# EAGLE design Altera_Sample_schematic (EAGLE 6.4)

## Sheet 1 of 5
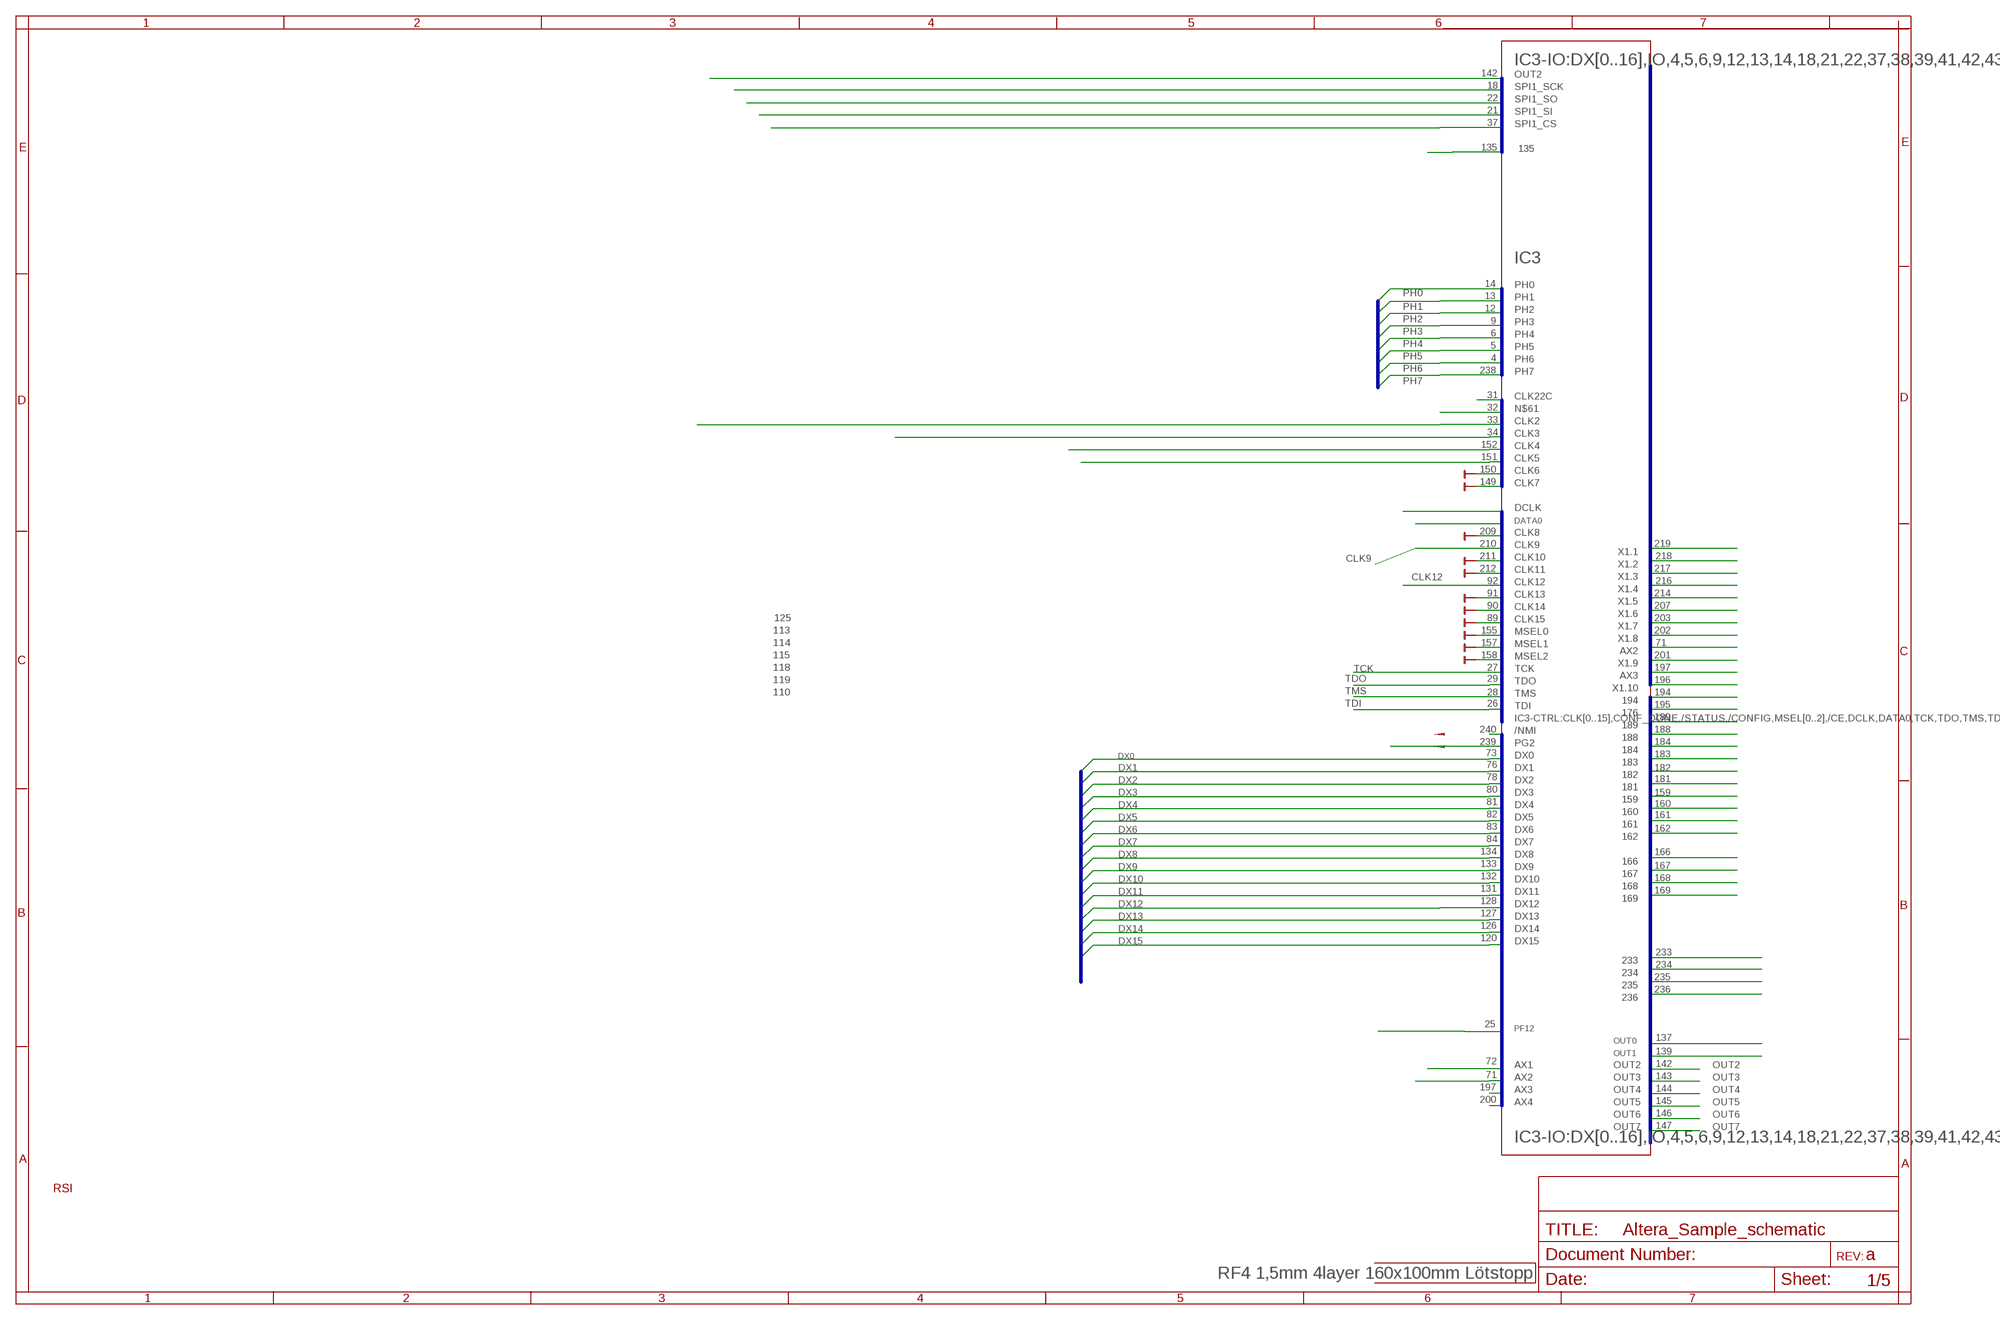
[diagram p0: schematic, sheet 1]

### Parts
PCB  RF4 1,5mm 4layer 160x100mm Lötstopp  PCB  [PCB]

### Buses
DATA:D[0..15]
SPI1:CS,SCK,SI,SO,PH[0..7]
IC3-IO:DX[0..16],IO,4,5,6,9,12,13,14,18,21,22,37,38,39,41,42,43,44,45,46,49,50,51,52,55,56,57,63,64,65,68,69,70,71,72,73,76,78,80,81,82,83,84,87,88,93,94,95,98,99,100,103,106,107,108,109,110,111,112,113,114,117,118,119,120,126,127,128,131,132,133,134,135,137,139,142,148,159,160,161,162,164,166,167,168,169,171,173,176,177,181,182,183,184,185,186,187,188,189,194,195,196,197,200,201,202,203,207,214,216,217,218,219,221,223,224,226,230,231,232,233,234,235,236,237,238,239,240
IC3-CTRL:CLK[0..15],CONF_DONE,/STATUS,/CONFIG,MSEL[0..2],/CE,DCLK,DATA0,TCK,TDO,TMS,TDI
IC3-PH:PH[0..7]

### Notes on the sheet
- 142
- 18
- 22
- 21
- 37
- 135
- IC3
- 14
- 13
- 12
- 9
- 6
- 5
- 4
- 238
- 31
- 32
- 33
- 34
- 152
- 151
- 150
- 149
- 209
- 210 | 219
- 211 | 218
- 212 | 217
- 92 | 216
- 91 | 214
- 90 | 207
- 125 | 89 | 203
- 113 | 155 | 202
- 114 | 157 | 71
- 115 | 158 | 201
- 118 | 27 | 197
- 119 | 29 | 196
- 110 | 28 | 194
- 26 | 195
- 189
- 240 | 188
- 239 | 184
- 73 | 183
- 76
- 182
- 78 | 181
- 80
- 159
- 81 | 160
- 82 | 161
- 83 | 162
- 84
- 134 | 166
- 133 | 167
- 132 | 168
- 131 | 169
- 128
- 127
- 126
- 120
- 233
- 234
- 235
- 236
- 25
- 137
- 139
- 72 | 142
- 71 | 143
- 197 | 144
- 200 | 145
- 146
- 147
- RSI

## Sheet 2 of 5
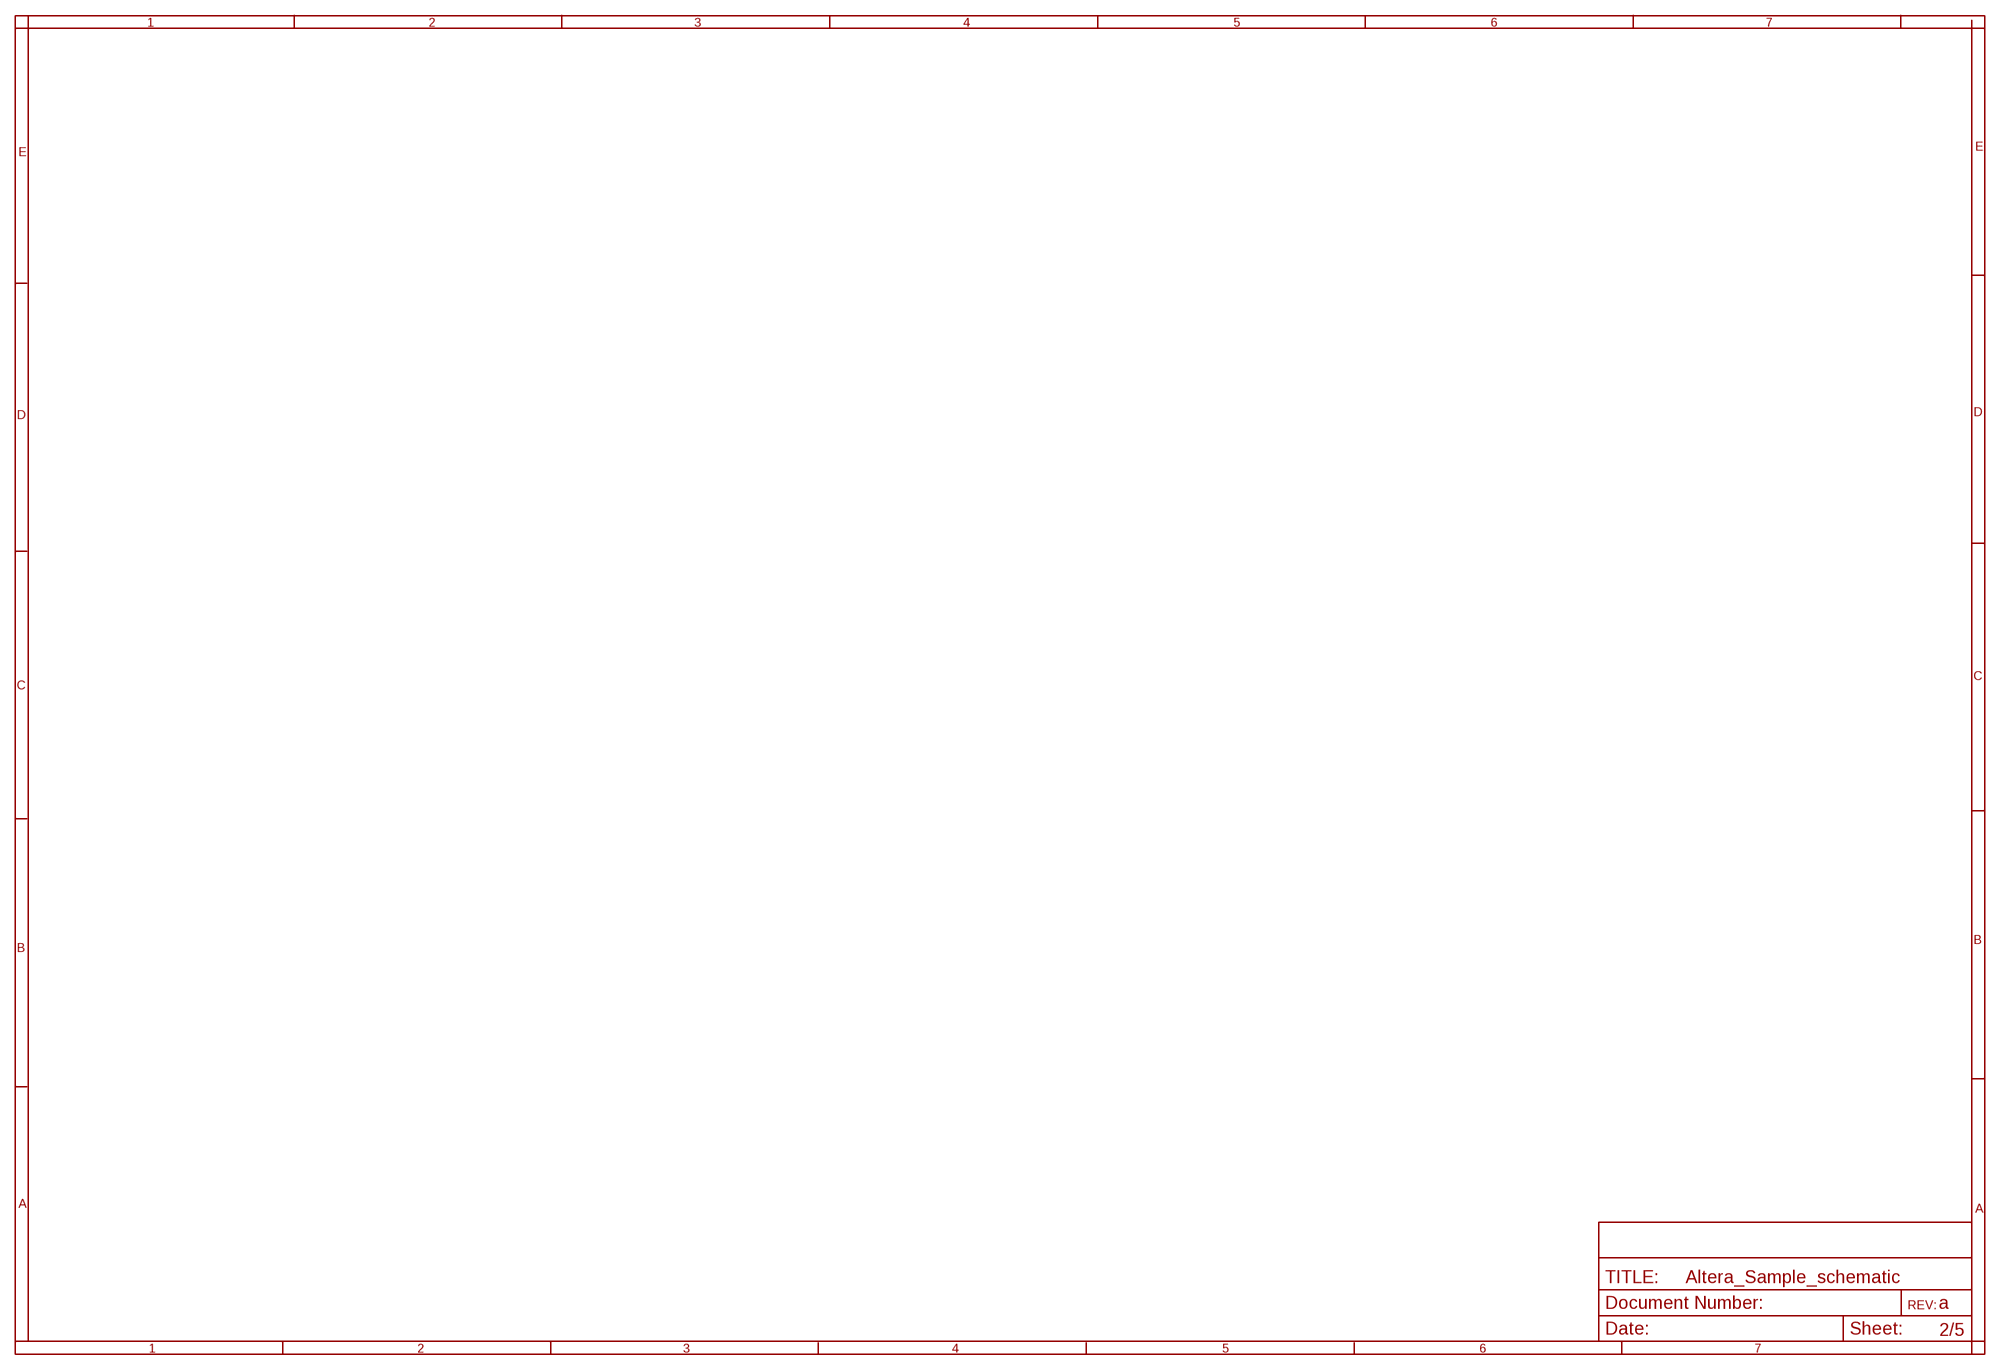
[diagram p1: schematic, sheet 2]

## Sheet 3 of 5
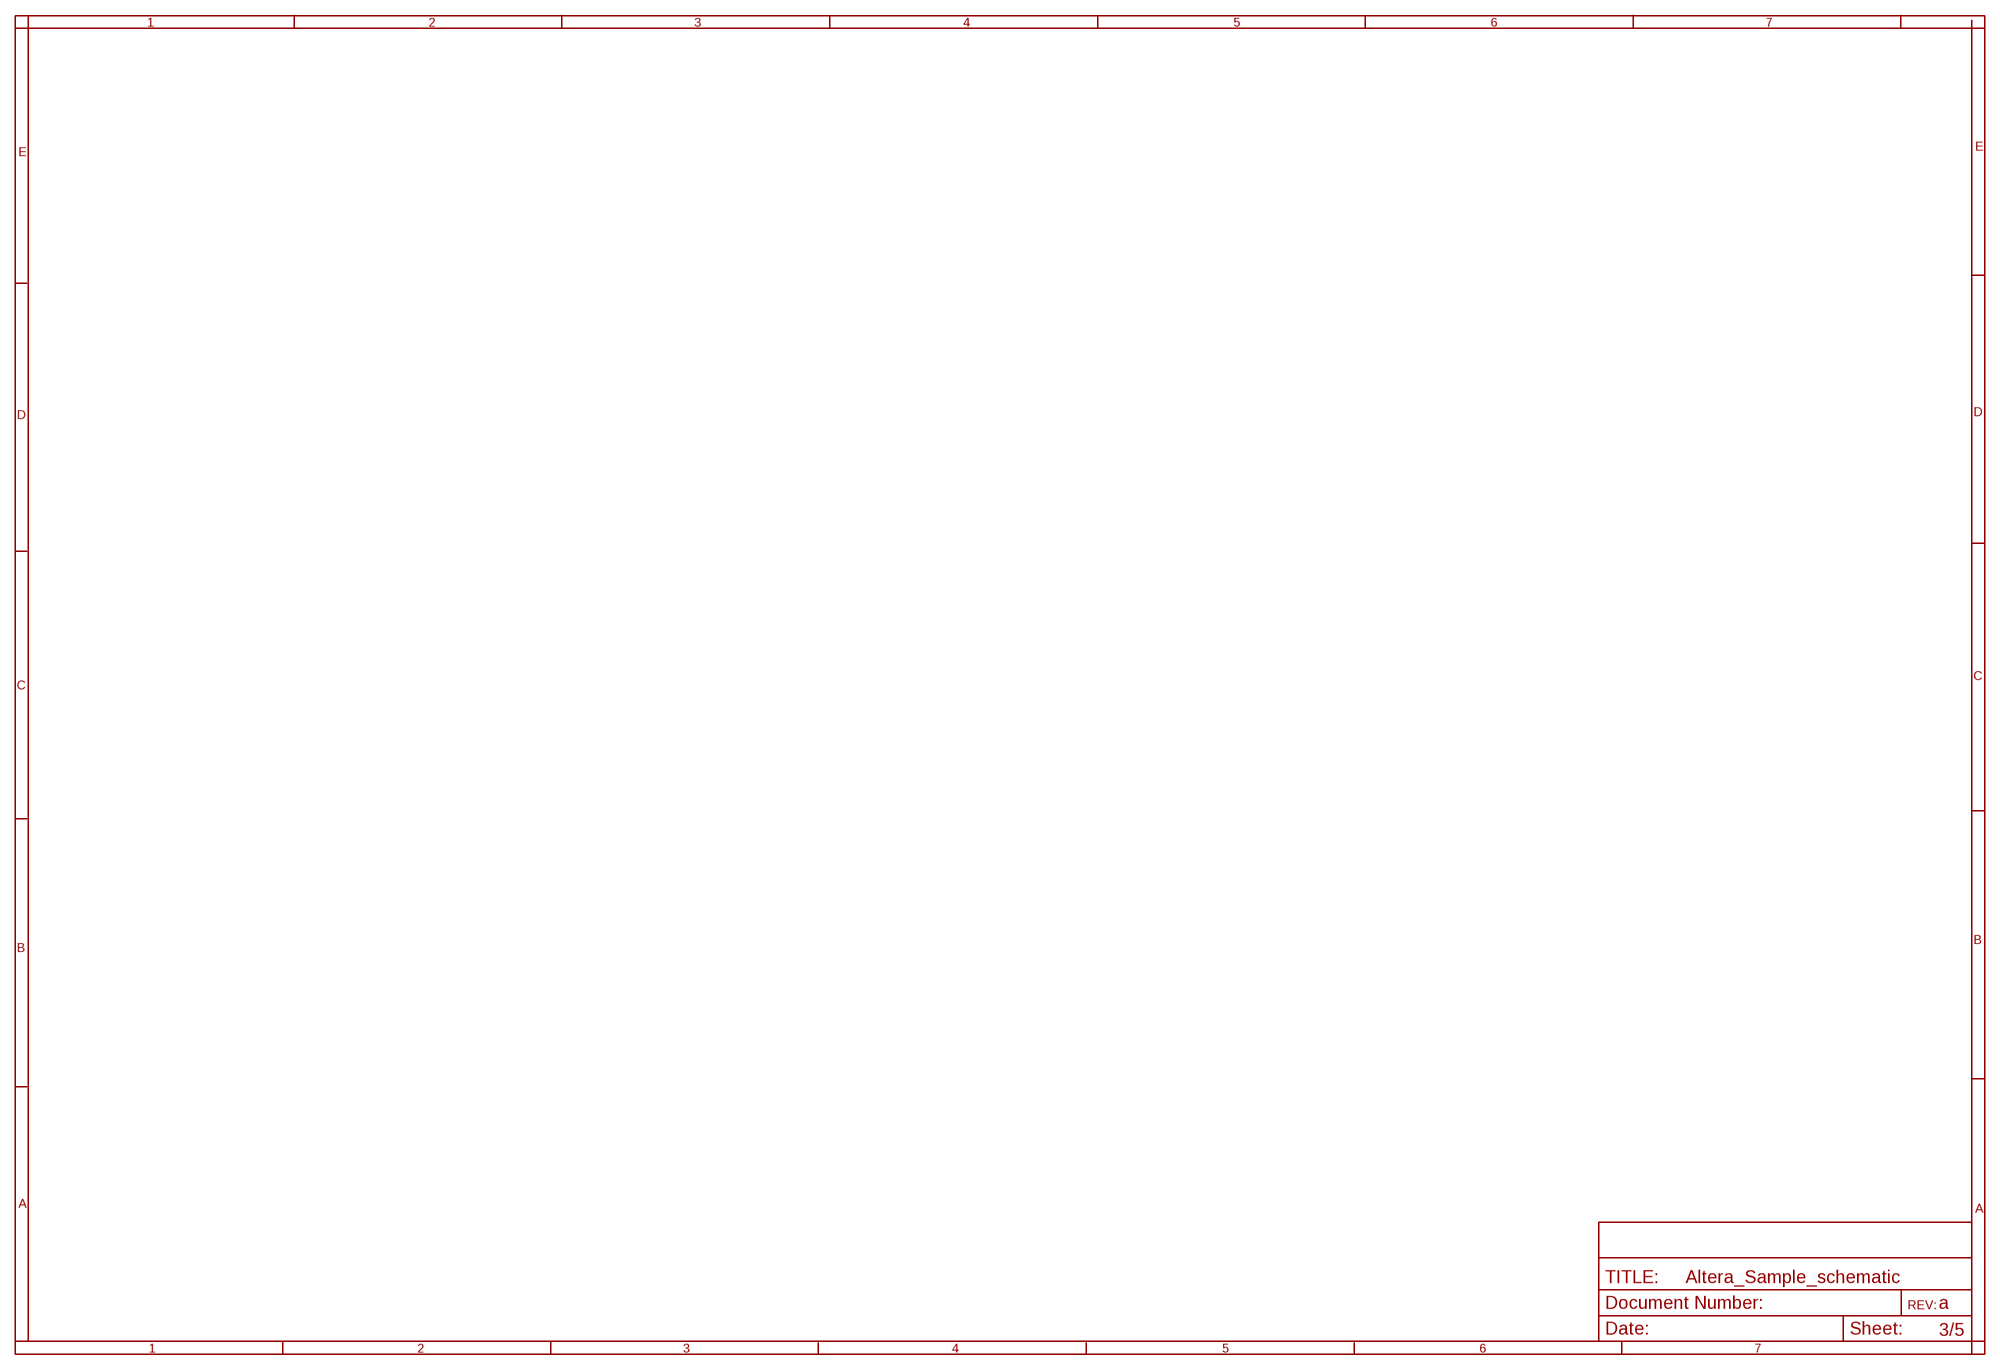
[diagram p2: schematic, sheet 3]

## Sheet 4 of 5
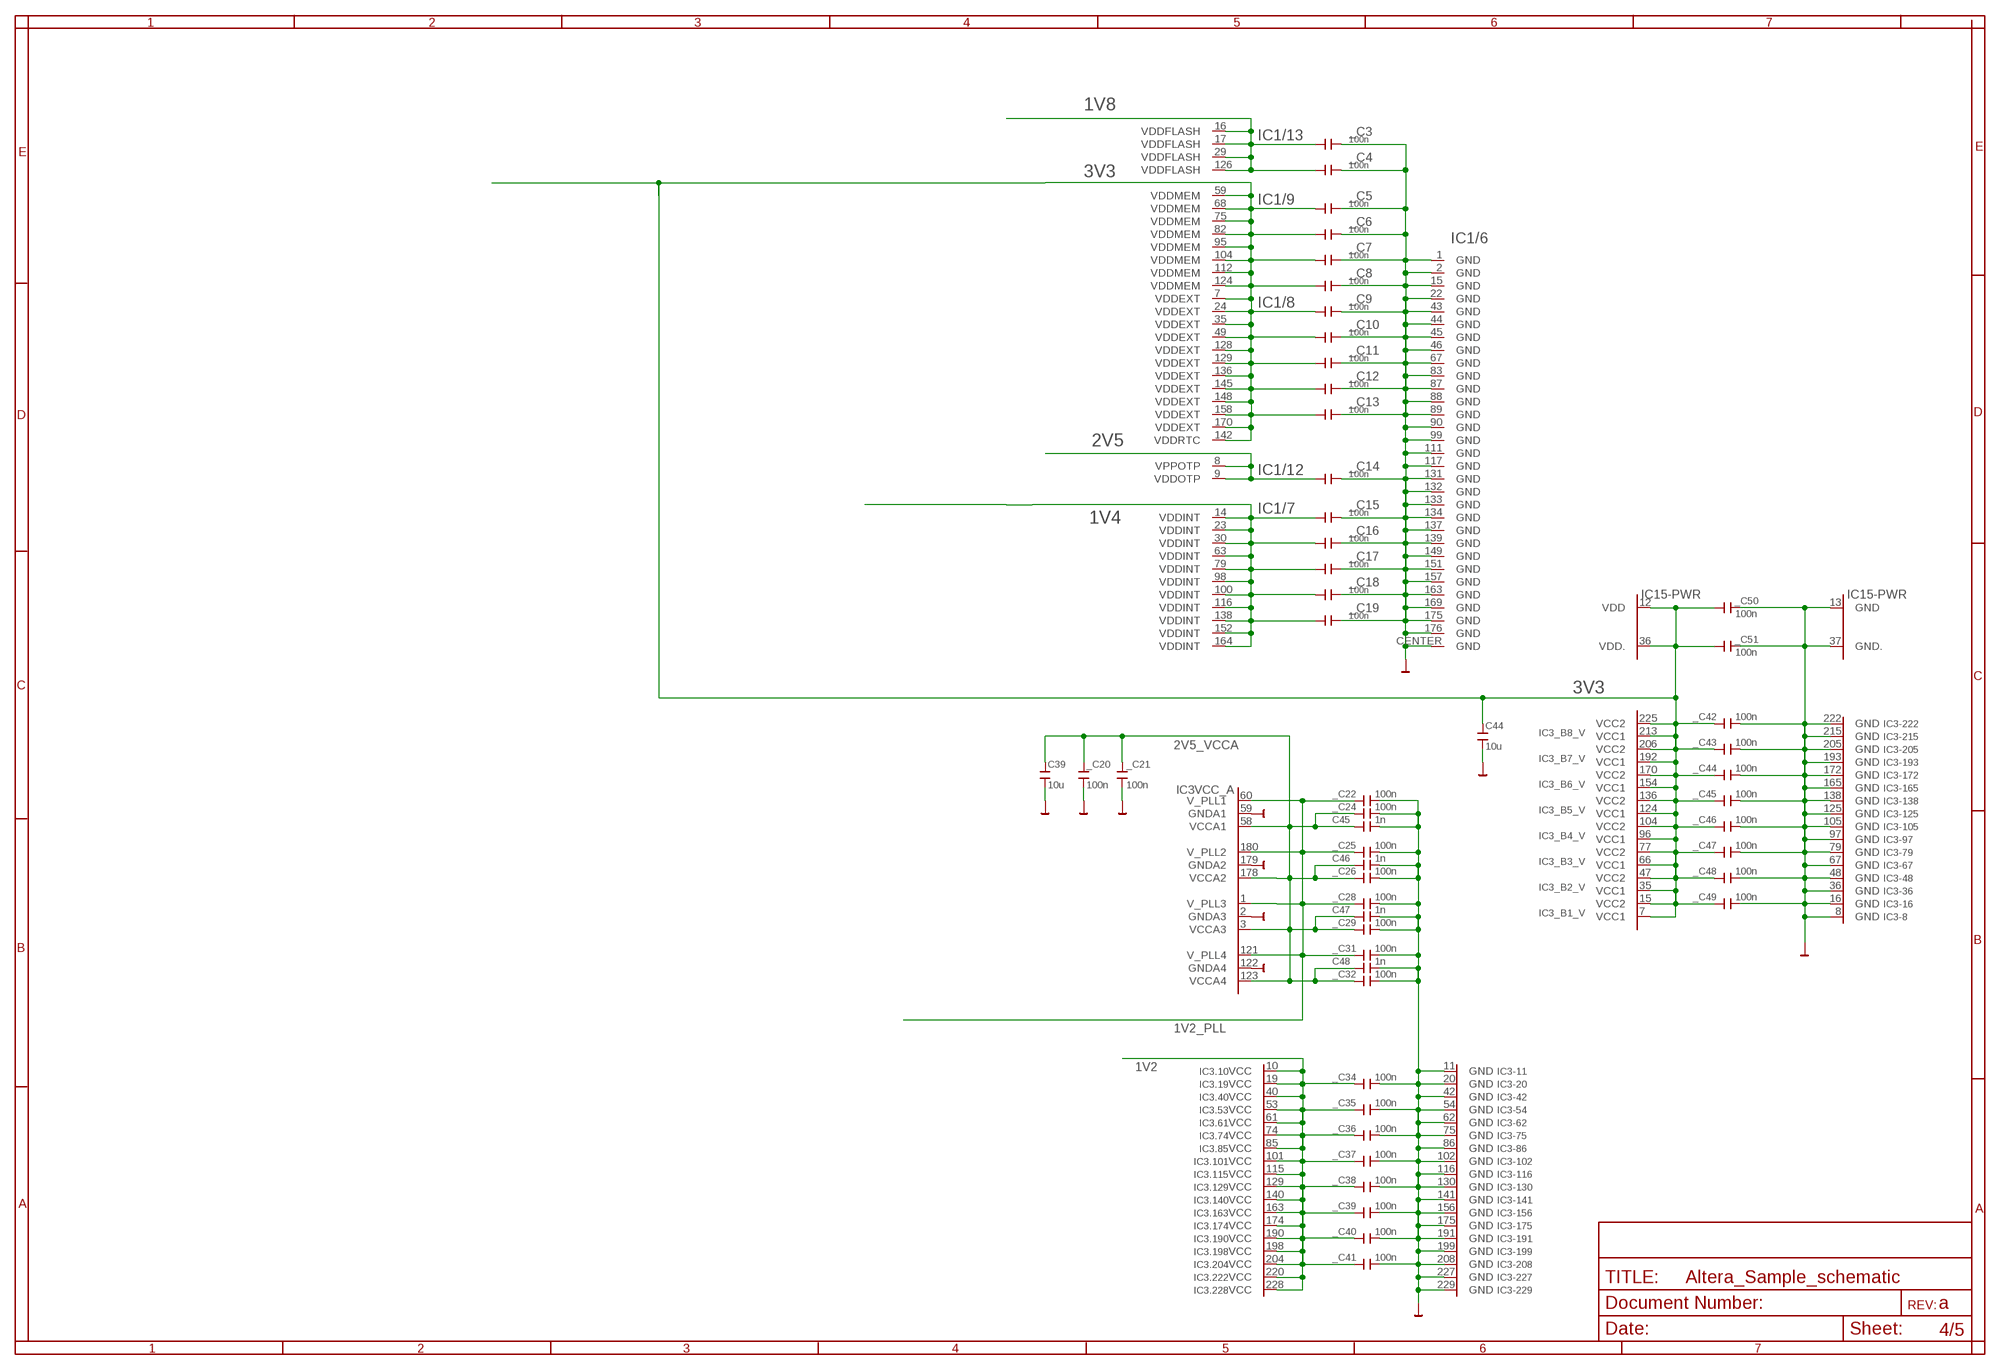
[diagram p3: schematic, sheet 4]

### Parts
_C3  100n  C-EUC0805  [C0805]
_C4  100n  C-EUC0805  [C0805]
_C5  100n  C-EUC0805  [C0805]
_C6  100n  C-EUC0805  [C0805]
_C7  100n  C-EUC0805  [C0805]
_C8  100n  C-EUC0805  [C0805]
_C9  100n  C-EUC0805  [C0805]
_C10  100n  C-EUC0805  [C0805]
_C11  100n  C-EUC0805  [C0805]
_C12  100n  C-EUC0805  [C0805]
_C13  100n  C-EUC0805  [C0805]
_C14  100n  C-EUC0805  [C0805]
_C15  100n  C-EUC0805  [C0805]
_C16  100n  C-EUC0805  [C0805]
_C17  100n  C-EUC0805  [C0805]
_C18  100n  C-EUC0805  [C0805]
_C19  100n  C-EUC0805  [C0805]
_C20  100n  C-EUC0805  [C0805]
_C21  100n  C-EUC0805  [C0805]
_C22  100n  C-EUC0805  [C0805]
_C24  100n  C-EUC0805  [C0805]
_C25  100n  C-EUC0805  [C0805]
_C26  100n  C-EUC0805  [C0805]
_C28  100n  C-EUC0805  [C0805]
_C29  100n  C-EUC0805  [C0805]
_C31  100n  C-EUC0805  [C0805]
_C32  100n  C-EUC0805  [C0805]
_C34  100n  C-EUC0805  [C0805]
_C35  100n  C-EUC0805  [C0805]
_C36  100n  C-EUC0805  [C0805]
_C37  100n  C-EUC0805  [C0805]
_C38  100n  C-EUC0805  [C0805]
_C39  100n  C-EUC0805  [C0805]
_C40  100n  C-EUC0805  [C0805]
_C41  100n  C-EUC0805  [C0805]
_C42  100n  C-EUC0805  [C0805]
_C43  100n  C-EUC0805  [C0805]
_C44  100n  C-EUC0805  [C0805]
_C45  100n  C-EUC0805  [C0805]
_C46  100n  C-EUC0805  [C0805]
_C47  100n  C-EUC0805  [C0805]
_C48  100n  C-EUC0805  [C0805]
_C49  100n  C-EUC0805  [C0805]
_C50  100n  C-EUC0805  [C0805]
_C51  100n  C-EUC0805  [C0805]
C39  10u  C-EUC1210K  [C1210K]
C44  10u  C-EUC1210K  [C1210K]
C45  1n  C-EUC0805  [C0805]
C46  1n  C-EUC0805  [C0805]
C47  1n  C-EUC0805  [C0805]
C48  1n  C-EUC0805  [C0805]
IC1  ADSP-BF514_PART  [LQFP-176+GND]
IC3  EP3C25-Q240-IO131  [PQFP240]
IC15  IS62WV102416ALL  [TSOP1-12X20]

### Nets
1V2: _C34.2 _C35.2 _C36.2 _C37.2 _C38.2 _C39.2 _C40.2 _C41.2 IC3.10(.10:VCC) IC3.19(.19:VCC) IC3.40(.40:VCC) IC3.53(.53:VCC) IC3.61(.61:VCC) IC3.74(.74:VCC) IC3.85(.85:VCC) IC3.101(.101:VCC) IC3.115(.115:VCC) IC3.129(.129:VCC) IC3.140(.140:VCC) IC3.163(.163:VCC) IC3.174(.174:VCC) IC3.190(.190:VCC) IC3.198(.198:VCC) IC3.204(.204:VCC) IC3.220(.222:VCC) IC3.228(.228:VCC)
1V2_PLL: _C22.2 _C25.2 _C28.2 _C31.2 IC3.1(VCC_A:V_PLL3) IC3.60(VCC_A:V_PLL1) IC3.121(VCC_A:V_PLL4) IC3.180(VCC_A:V_PLL2)
1V4: _C15.1 _C16.1 _C17.1 _C18.1 _C19.1 IC1.14(/7:VDDINT) IC1.23(/7:VDDINT) IC1.30(/7:VDDINT) IC1.63(/7:VDDINT) IC1.79(/7:VDDINT) IC1.98(/7:VDDINT) IC1.100(/7:VDDINT) IC1.116(/7:VDDINT) IC1.138(/7:VDDINT) IC1.152(/7:VDDINT) IC1.164(/7:VDDINT)
1V8: _C3.1 _C4.1 IC1.16(/13:VDDFLASH) IC1.17(/13:VDDFLASH) IC1.29(/13:VDDFLASH) IC1.126(/13:VDDFLASH)
2V5: _C14.1 IC1.8(/12:VPPOTP) IC1.9(/12:VDDOTP)
2V5_VCCA: _C20.2 _C21.2 _C24.2 _C26.2 _C29.2 _C32.2 C39.2 C45.2 C46.2 C47.2 C48.2 IC3.3(VCC_A:VCCA3) IC3.58(VCC_A:VCCA1) IC3.123(VCC_A:VCCA4) IC3.178(VCC_A:VCCA2)
3V3: _C5.1 _C6.1 _C7.1 _C8.1 _C9.1 _C10.1 _C11.1 _C12.1 _C13.1 _C42.2 _C43.2 _C44.2 _C45.2 _C46.2 _C47.2 _C48.2 _C49.2 _C50.1 _C51.1 C44.2 IC1.7(/8:VDDEXT) IC1.24(/8:VDDEXT) IC1.35(/8:VDDEXT) IC1.49(/8:VDDEXT) IC1.59(/9:VDDMEM) IC1.68(/9:VDDMEM) IC1.75(/9:VDDMEM) IC1.82(/9:VDDMEM) IC1.95(/9:VDDMEM) IC1.104(/9:VDDMEM) IC1.112(/9:VDDMEM) IC1.124(/9:VDDMEM) IC1.128(/8:VDDEXT) IC1.129(/8:VDDEXT) IC1.136(/8:VDDEXT) IC1.142(/12:VDDRTC) IC1.145(/8:VDDEXT) IC1.148(/8:VDDEXT) IC1.158(/8:VDDEXT) IC1.170(/8:VDDEXT) IC3.7(_B1_V:VCC1) IC3.15(_B1_V:VCC2) IC3.35(_B2_V:VCC1) IC3.47(_B2_V:VCC2) IC3.66(_B3_V:VCC1) IC3.77(_B3_V:VCC2) IC3.96(_B4_V:VCC1) IC3.104(_B4_V:VCC2) IC3.124(_B5_V:VCC1) IC3.136(_B5_V:VCC2) IC3.154(_B6_V:VCC1) IC3.170(_B6_V:VCC2) IC3.192(_B7_V:VCC1) IC3.206(_B7_V:VCC2) IC3.213(_B8_V:VCC1) IC3.225(_B8_V:VCC2) IC15.12(-PWR:VDD) IC15.36(-PWR:VDD.)
GND: _C3.2 _C4.2 _C5.2 _C6.2 _C7.2 _C8.2 _C9.2 _C10.2 _C11.2 _C12.2 _C13.2 _C14.2 _C15.2 _C16.2 _C17.2 _C18.2 _C19.2 _C20.1 _C21.1 _C22.1 _C24.1 _C25.1 _C26.1 _C28.1 _C29.1 _C31.1 _C32.1 _C34.1 _C35.1 _C36.1 _C37.1 _C38.1 _C39.1 _C40.1 _C41.1 _C42.1 _C43.1 _C44.1 _C45.1 _C46.1 _C47.1 _C48.1 _C49.1 _C50.2 _C51.2 C39.1 C44.1 C45.1 C46.1 C47.1 C48.1 IC1.1(/6:GND) IC1.2(/6:GND) IC1.15(/6:GND) IC1.22(/6:GND) IC1.43(/6:GND) IC1.44(/6:GND) IC1.45(/6:GND) IC1.46(/6:GND) IC1.67(/6:GND) IC1.83(/6:GND) IC1.87(/6:GND) IC1.88(/6:GND) IC1.89(/6:GND) IC1.90(/6:GND) IC1.99(/6:GND) IC1.111(/6:GND) IC1.117(/6:GND) IC1.131(/6:GND) IC1.132(/6:GND) IC1.133(/6:GND) IC1.134(/6:GND) IC1.137(/6:GND) IC1.139(/6:GND) IC1.149(/6:GND) IC1.151(/6:GND) IC1.157(/6:GND) IC1.163(/6:GND) IC1.169(/6:GND) IC1.175(/6:GND) IC1.176(/6:GND) IC1.CENTER(/6:GND) IC3.2(VCC_A:GNDA3) IC3.8(-8:GND) IC3.11(-11:GND) IC3.16(-16:GND) IC3.20(-20:GND) IC3.36(-36:GND) IC3.42(-42:GND) IC3.48(-48:GND) IC3.54(-54:GND) IC3.59(VCC_A:GNDA1) IC3.62(-62:GND) IC3.67(-67:GND) IC3.75(-75:GND) IC3.79(-79:GND) IC3.86(-86:GND) IC3.97(-97:GND) IC3.102(-102:GND) IC3.105(-105:GND) IC3.116(-116:GND) IC3.122(VCC_A:GNDA4) IC3.125(-125:GND) IC3.130(-130:GND) IC3.138(-138:GND) IC3.141(-141:GND) IC3.156(-156:GND) IC3.165(-165:GND) IC3.172(-172:GND) IC3.175(-175:GND) IC3.179(VCC_A:GNDA2) IC3.191(-191:GND) IC3.193(-193:GND) IC3.199(-199:GND) IC3.205(-205:GND) IC3.208(-208:GND) IC3.215(-215:GND) IC3.222(-222:GND) IC3.227(-227:GND) IC3.229(-229:GND) IC15.13(-PWR:GND) IC15.37(-PWR:GND.) ; also sheet 5
Unconnected: IC1.3(/3:PF9) IC1.4(/3:PF8) IC1.5(/3:PF7) IC1.6(/3:PF6) IC1.10(/3:PF5) IC1.11(/3:PF4) IC1.12(/3:PF3) IC1.13(/3:PF2) IC1.18(/3:PF1) IC1.19(/3:PF0) IC1.20(/4:PG15) IC1.21(/4:PG14) IC1.25(/4:PG13) IC1.26(/4:PG12) IC1.27(/4:PG11) IC1.28(/4:PG10) IC1.31(/4:PG9) IC1.32(/4:PG8) IC1.33(/4:PG7) IC1.34(/4:PG6) IC1.36(/4:PG5) IC1.37(/4:PG4) IC1.38(/4:PG3) IC1.39(/4:PG2) IC1.47(/4:PG1) IC1.48(/4:PG0) IC1.50(/11:TDO) IC1.51(/11:/EMU) IC1.52(/11:TDI) IC1.53(/11:TCK) IC1.54(/11:/TRST) IC1.55(/11:TMS) IC1.56(/2:D15) IC1.57(/2:D14) IC1.58(/2:D13) IC1.60(/2:D12) IC1.61(/2:D11) IC1.62(/2:D10) IC1.64(/2:D9) IC1.65(/2:D8) IC1.66(/2:D7) IC1.69(/2:D6) IC1.70(/2:D5) IC1.71(/2:D4) IC1.72(/2:D3) IC1.73(/2:D2) IC1.74(/2:D1) IC1.76(/2:D0) IC1.77(/1:A19) IC1.78(/1:A18) IC1.80(/1:A17) IC1.81(/1:A16) IC1.84(/1:A15) IC1.85(/1:A14) IC1.86(/1:A13) IC1.91(/1:A12) IC1.92(/1:A11) IC1.93(/1:A10) IC1.94(/1:A9) IC1.96(/1:A8) IC1.97(/1:A7) IC1.101(/1:A6) IC1.102(/1:A5) IC1.103(/1:A4) IC1.105(/1:A3) IC1.106(/1:A2) IC1.107(/1:A1) IC1.108(/11:/ABE1) IC1.109(/11:/ABE0) IC1.110(/11:SA10) IC1.113(/11:/SWE) IC1.114(/11:/SCAS) IC1.115(/11:/SRAS) IC1.118(/11:/SMS) IC1.119(/11:SCKE) IC1.120(/11:/AMS1) IC1.121(/11:/ARE) IC1.122(/11:/AWE) IC1.123(/11:/AMS0) IC1.125(/11:CLKOUT) IC1.127(/11:NC) IC1.130(/11:EXT_WAKE) IC1.135(/11:/PG) IC1.140(/11:RTXO) IC1.141(/11:RTXI) IC1.143(/11:CLKIN) IC1.144(/11:XTAL) IC1.146(/11:/RESET) IC1.147(/11:/NMI) IC1.150(/11:CLKBUF) IC1.153(/5:PH7) IC1.154(/5:PH6) IC1.155(/5:PH5) IC1.156(/5:PH4) IC1.159(/5:PH3) IC1.160(/5:PH2) IC1.161(/5:PH1) IC1.162(/5:PH0) IC1.165(/3:PF15) IC1.166(/3:PF14) IC1.167(/3:PF13) IC1.168(/3:PF12) IC1.171(/3:PF11) IC1.172(/11:SDA) IC1.173(/11:SCL) IC1.174(/3:PF10)

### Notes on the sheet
- IC1/13
- IC1/9
- IC1/6
- IC1/8
- IC1/12
- IC1/7

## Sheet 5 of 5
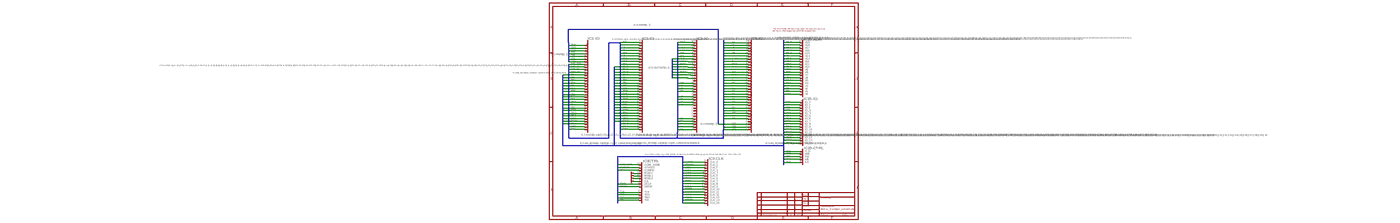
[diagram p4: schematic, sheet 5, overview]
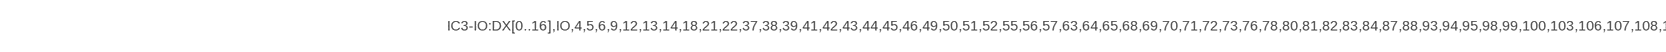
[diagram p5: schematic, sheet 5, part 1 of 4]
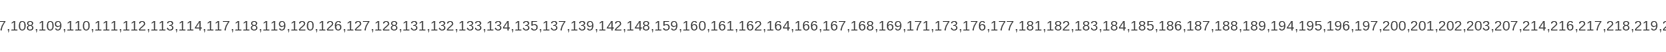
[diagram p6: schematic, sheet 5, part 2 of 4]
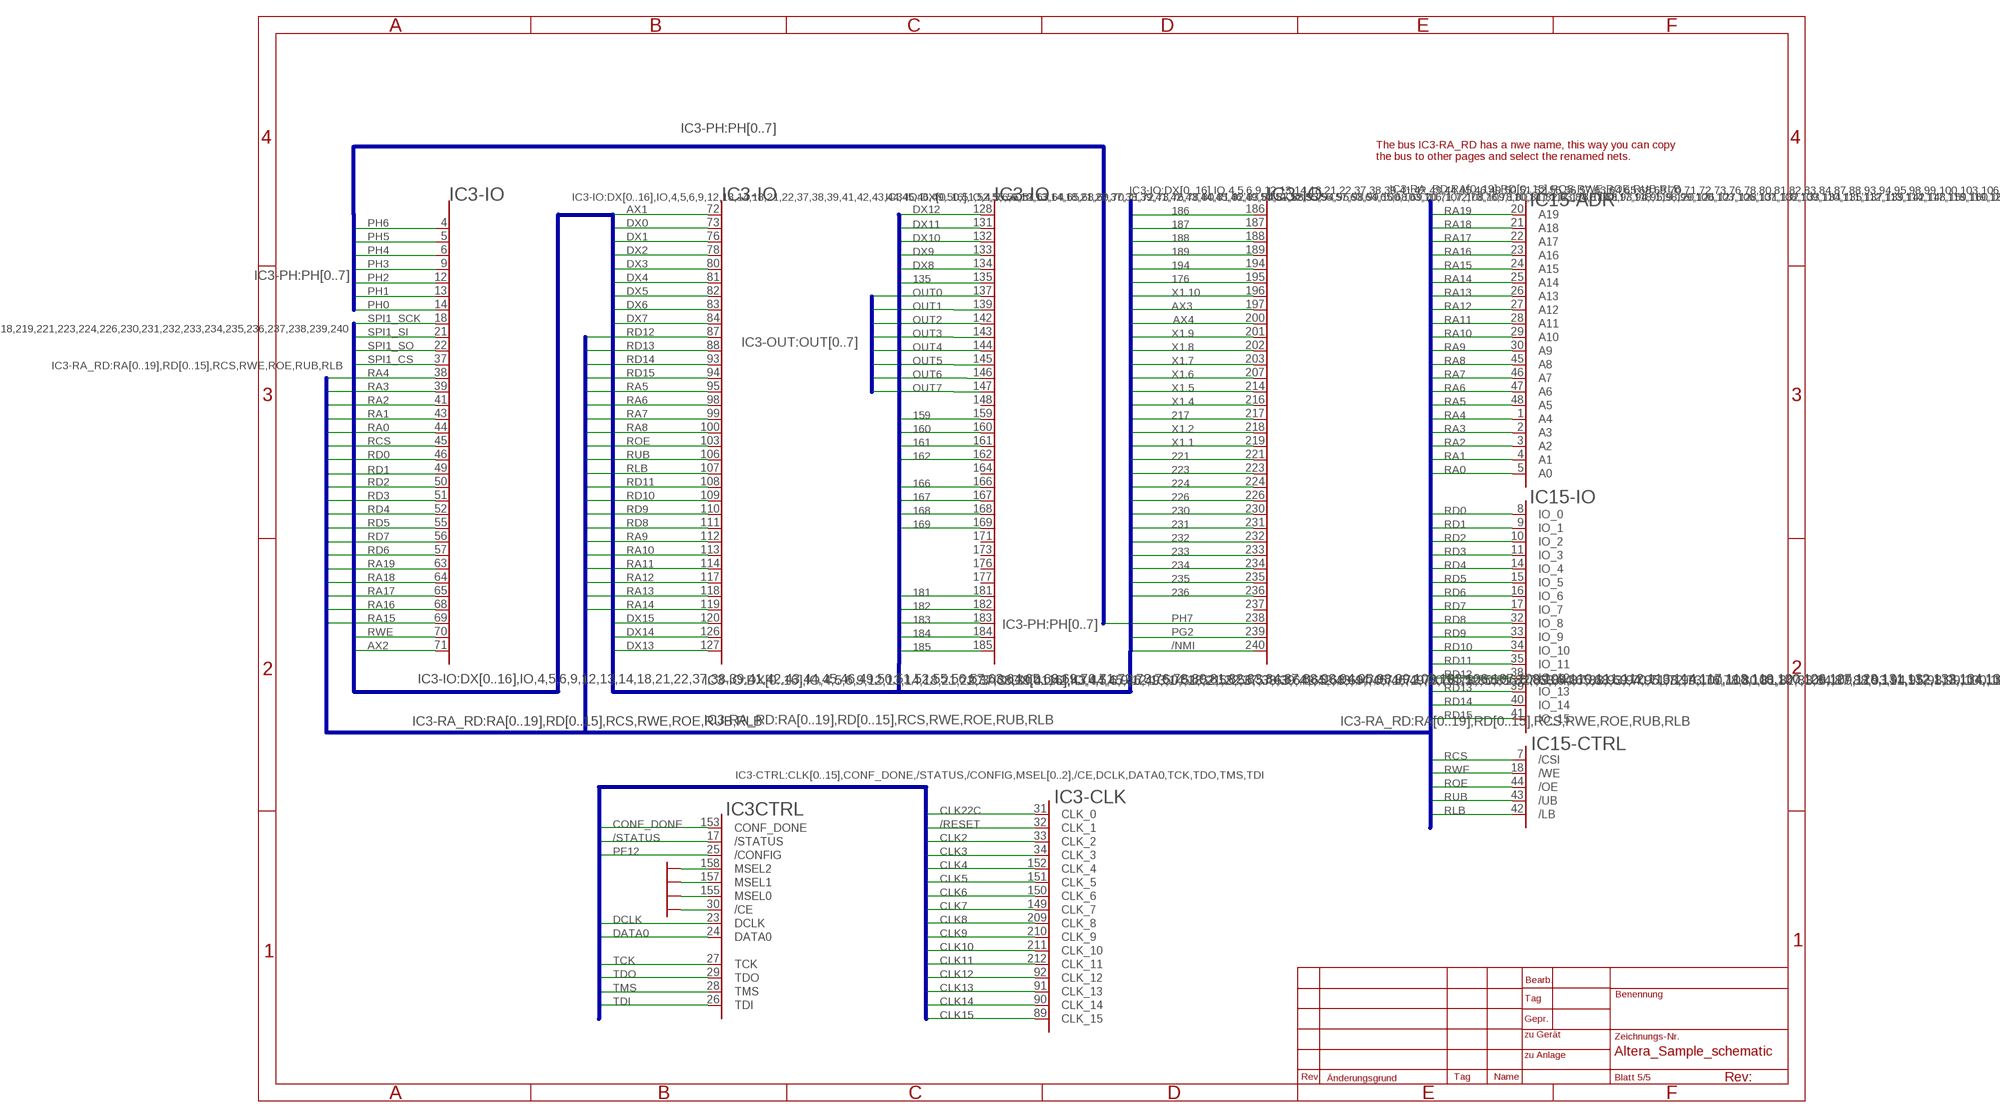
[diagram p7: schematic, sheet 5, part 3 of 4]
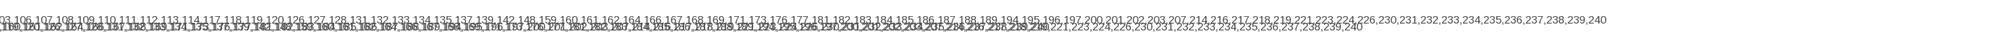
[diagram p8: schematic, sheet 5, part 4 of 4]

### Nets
135: IC3.135(IO_71) ; also sheet 1
159: IC3.159(IO_81) ; also sheet 1
160: IC3.160(IO_82) ; also sheet 1
161: IC3.161(IO_83) ; also sheet 1
162: IC3.162(IO_84) ; also sheet 1
166: IC3.166(IO_86) ; also sheet 1
167: IC3.167(IO_87) ; also sheet 1
168: IC3.168(IO_88) ; also sheet 1
169: IC3.169(IO_89) ; also sheet 1
176: IC3.195(IO_104) ; also sheet 1
181: IC3.181(IO_94) ; also sheet 1
182: IC3.182(IO_95) ; also sheet 1
183: IC3.183(IO_96) ; also sheet 1
184: IC3.184(IO_97) ; also sheet 1
185: IC3.185(IO_98)
186: IC3.186(IO_99)
187: IC3.187(IO_100)
188: IC3.188(IO_101) ; also sheet 1
189: IC3.189(IO_102) ; also sheet 1
194: IC3.194(IO_103) ; also sheet 1
217: IC3.217(IO_114)
221: IC3.221(IO_117)
223: IC3.223(IO_118)
224: IC3.224(IO_119)
226: IC3.226(IO_120)
230: IC3.230(IO_121)
231: IC3.231(IO_122)
232: IC3.232(IO_123)
233: IC3.233(IO_124) ; also sheet 1
234: IC3.234(IO_125) ; also sheet 1
235: IC3.235(IO_126) ; also sheet 1
236: IC3.236(IO_127) ; also sheet 1
/NMI: IC3.240(IO_131) ; also sheet 1
/RESET: IC3.32(-CLK:CLK_1)
/STATUS: IC3.17(CTRL:/STATUS)
AX1: IC3.72(IO_33) ; also sheet 1
AX2: IC3.71(IO_32) ; also sheet 1
AX3: IC3.197(IO_106) ; also sheet 1
AX4: IC3.200(IO_107) ; also sheet 1
CLK2: IC3.33(-CLK:CLK_2) ; also sheet 1
CLK3: IC3.34(-CLK:CLK_3) ; also sheet 1
CLK4: IC3.152(-CLK:CLK_4) ; also sheet 1
CLK5: IC3.151(-CLK:CLK_5) ; also sheet 1
CLK6: IC3.150(-CLK:CLK_6) ; also sheet 1
CLK7: IC3.149(-CLK:CLK_7) ; also sheet 1
CLK8: IC3.209(-CLK:CLK_8) ; also sheet 1
CLK9: IC3.210(-CLK:CLK_9) ; also sheet 1
CLK10: IC3.211(-CLK:CLK_10) ; also sheet 1
CLK11: IC3.212(-CLK:CLK_11) ; also sheet 1
CLK12: IC3.92(-CLK:CLK_12) ; also sheet 1
CLK13: IC3.91(-CLK:CLK_13) ; also sheet 1
CLK14: IC3.90(-CLK:CLK_14) ; also sheet 1
CLK15: IC3.89(-CLK:CLK_15) ; also sheet 1
CLK22C: IC3.31(-CLK:CLK_0) ; also sheet 1
CONF_DONE: IC3.153(CTRL:CONF_DONE)
DATA0: IC3.24(CTRL:DATA0) ; also sheet 1
DCLK: IC3.23(CTRL:DCLK) ; also sheet 1
DX0: IC3.73(IO_34) ; also sheet 1
DX1: IC3.76(IO_35) ; also sheet 1
DX2: IC3.78(IO_36) ; also sheet 1
DX3: IC3.80(IO_37) ; also sheet 1
DX4: IC3.81(IO_38) ; also sheet 1
DX5: IC3.82(IO_39) ; also sheet 1
DX6: IC3.83(IO_40) ; also sheet 1
DX7: IC3.84(IO_41) ; also sheet 1
DX8: IC3.134(IO_70) ; also sheet 1
DX9: IC3.133(IO_69) ; also sheet 1
DX10: IC3.132(IO_68) ; also sheet 1
DX11: IC3.131(IO_67) ; also sheet 1
DX12: IC3.128(IO_66) ; also sheet 1
DX13: IC3.127(IO_65) ; also sheet 1
DX14: IC3.126(IO_64) ; also sheet 1
DX15: IC3.120(IO_63) ; also sheet 1
GND: IC3.30(CTRL:/CE) IC3.155(CTRL:MSEL0) IC3.157(CTRL:MSEL1) IC3.158(CTRL:MSEL2) ; also sheet 4
OUT0: IC3.137(IO_72) ; also sheet 1
OUT1: IC3.139(IO_73) ; also sheet 1
OUT2: IC3.142(IO_74) ; also sheet 1
OUT3: IC3.143(IO_75) ; also sheet 1
OUT4: IC3.144(IO_76) ; also sheet 1
OUT5: IC3.145(IO_77) ; also sheet 1
OUT6: IC3.146(IO_78) ; also sheet 1
OUT7: IC3.147(IO_79) ; also sheet 1
PF12: IC3.25(CTRL:/CONFIG) ; also sheet 1
PG2: IC3.239(IO_130) ; also sheet 1
PH0: IC3.14(IO_7) ; also sheet 1
PH1: IC3.13(IO_6) ; also sheet 1
PH2: IC3.12(IO_5) ; also sheet 1
PH3: IC3.9(IO_4) ; also sheet 1
PH4: IC3.6(IO_3) ; also sheet 1
PH5: IC3.5(IO_2) ; also sheet 1
PH6: IC3.4(IO_1) ; also sheet 1
PH7: IC3.238(IO_129) ; also sheet 1
RA0: IC3.44(IO_16) IC15.5(-ADR:A0)
RA1: IC3.43(IO_15) IC15.4(-ADR:A1)
RA2: IC3.41(IO_14) IC15.3(-ADR:A2)
RA3: IC3.39(IO_13) IC15.2(-ADR:A3)
RA4: IC3.38(IO_12) IC15.1(-ADR:A4)
RA5: IC3.95(IO_46) IC15.48(-ADR:A5)
RA6: IC3.98(IO_47) IC15.47(-ADR:A6)
RA7: IC3.99(IO_48) IC15.46(-ADR:A7)
RA8: IC3.100(IO_49) IC15.45(-ADR:A8)
RA9: IC3.112(IO_57) IC15.30(-ADR:A9)
RA10: IC3.113(IO_58) IC15.29(-ADR:A10)
RA11: IC3.114(IO_59) IC15.28(-ADR:A11)
RA12: IC3.117(IO_60) IC15.27(-ADR:A12)
RA13: IC3.118(IO_61) IC15.26(-ADR:A13)
RA14: IC3.119(IO_62) IC15.25(-ADR:A14)
RA15: IC3.69(IO_30) IC15.24(-ADR:A15)
RA16: IC3.68(IO_29) IC15.23(-ADR:A16)
RA17: IC3.65(IO_28) IC15.22(-ADR:A17)
RA18: IC3.64(IO_27) IC15.21(-ADR:A18)
RA19: IC3.63(IO_26) IC15.20(-ADR:A19)
RCS: IC3.45(IO_17) IC15.7(-CTRL:/CSI)
RD0: IC3.46(IO_18) IC15.8(-IO:IO_0)
RD1: IC3.49(IO_19) IC15.9(-IO:IO_1)
RD2: IC3.50(IO_20) IC15.10(-IO:IO_2)
RD3: IC3.51(IO_21) IC15.11(-IO:IO_3)
RD4: IC3.52(IO_22) IC15.14(-IO:IO_4)
RD5: IC3.55(IO_23) IC15.15(-IO:IO_5)
RD6: IC3.57(IO_25) IC15.16(-IO:IO_6)
RD7: IC3.56(IO_24) IC15.17(-IO:IO_7)
RD8: IC3.111(IO_56) IC15.32(-IO:IO_8)
RD9: IC3.110(IO_55) IC15.33(-IO:IO_9)
RD10: IC3.109(IO_54) IC15.34(-IO:IO_10)
RD11: IC3.108(IO_53) IC15.35(-IO:IO_11)
RD12: IC3.87(IO_42) IC15.38(-IO:IO_12)
RD13: IC3.88(IO_43) IC15.39(-IO:IO_13)
RD14: IC3.93(IO_44) IC15.40(-IO:IO_14)
RD15: IC3.94(IO_45) IC15.41(-IO:IO_15)
RLB: IC3.107(IO_52) IC15.42(-CTRL:/LB)
ROE: IC3.103(IO_50) IC15.44(-CTRL:/OE)
RUB: IC3.106(IO_51) IC15.43(-CTRL:/UB)
RWE: IC3.70(IO_31) IC15.18(-CTRL:/WE)
SPI1_CS: IC3.37(IO_11) ; also sheet 1
SPI1_SCK: IC3.18(IO_8) ; also sheet 1
SPI1_SI: IC3.21(IO_9) ; also sheet 1
SPI1_SO: IC3.22(IO_10) ; also sheet 1
TCK: IC3.27(CTRL:TCK) ; also sheet 1
TDI: IC3.26(CTRL:TDI) ; also sheet 1
TDO: IC3.29(CTRL:TDO) ; also sheet 1
TMS: IC3.28(CTRL:TMS) ; also sheet 1
X1.1: IC3.219(IO_116) ; also sheet 1
X1.2: IC3.218(IO_115) ; also sheet 1
X1.4: IC3.216(IO_113) ; also sheet 1
X1.5: IC3.214(IO_112) ; also sheet 1
X1.6: IC3.207(IO_111) ; also sheet 1
X1.7: IC3.203(IO_110) ; also sheet 1
X1.8: IC3.202(IO_109) ; also sheet 1
X1.9: IC3.201(IO_108) ; also sheet 1
X1.10: IC3.196(IO_105) ; also sheet 1
Unconnected: IC3.148(IO_80) IC3.164(IO_85) IC3.171(IO_90) IC3.173(IO_91) IC3.176(IO_92) IC3.177(IO_93) IC3.237(IO_128)

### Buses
IC3-IO:DX[0..16],IO,4,5,6,9,12,13,14,18,21,22,37,38,39,41,42,43,44,45,46,49,50,51,52,55,56,57,63,64,65,68,69,70,71,72,73,76,78,80,81,82,83,84,87,88,93,94,95,98,99,100,103,106,107,108,109,110,111,112,113,114,117,118,119,120,126,127,128,131,132,133,134,135,137,139,142,148,159,160,161,162,164,166,167,168,169,171,173,176,177,181,182,183,184,185,186,187,188,189,194,195,196,197,200,201,202,203,207,214,216,217,218,219,221,223,224,226,230,231,232,233,234,235,236,237,238,239,240
IC3-CTRL:CLK[0..15],CONF_DONE,/STATUS,/CONFIG,MSEL[0..2],/CE,DCLK,DATA0,TCK,TDO,TMS,TDI
IC3-PH:PH[0..7]
IC3-OUT:OUT[0..7]
IC3-RA_RD:RA[0..19],RD[0..15],RCS,RWE,ROE,RUB,RLB

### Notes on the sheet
- The bus IC3-RA_RD has a nwe name, this way you can copy 
  the bus to other pages and select the renamed nets.
- IC3-IO | IC3-IO | IC3-IO | IC3-IO

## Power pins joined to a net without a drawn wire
BMODE0: IC1.42(/10:BMODE0)
BMODE1: IC1.41(/10:BMODE1)
BMODE2: IC1.40(/10:BMODE2)

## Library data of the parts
_C3-_C22 _C24-_C26 _C28 _C29 _C31 _C32 _C34-_C51 C39 C44-C48 = rcl:C-EU: CAPACITOR, European symbol
IC1 = sastec:ADSP-BF514_PART
IC3 = sastec:EP3C25-Q240-IO131: EPF10K30 FLEX 10K family; BUS-CTRL: -CTRL:CLK[0..15],CONF_DONE,/STATUS,/CONFIG,MSEL[0..2],/CE,DCLK,DATA0,TCK,TDO,TMS,TDI; BUS-IO: -IO:PIN#,4,5,6,9,12,13,14,18,21,22,37,38,39,41,42,43,44,45,46,49,50,51,52,55,56,57,63,64,65,68,69,70,71,72,73,76,78,80,81,82,83,84,87,88,93,94,95,98,99,100,103,106,107,108,109,110,111,112,113,114,117,118,119,120,126,127,128,131,132,133,134,135,137,139,142,148,159,160,161,162,164,166,167,168,169,171,173,176,177,181,182,183,184,185,186,187,188,189,194,195,196,197,200,201,202,203,207,214,216,217,218,219,221,223,224,226,230,231,232,233,234,235,236,237,238,239,240
IC15 = sastec:IS62WV102416ALL
PCB = frames:PCB

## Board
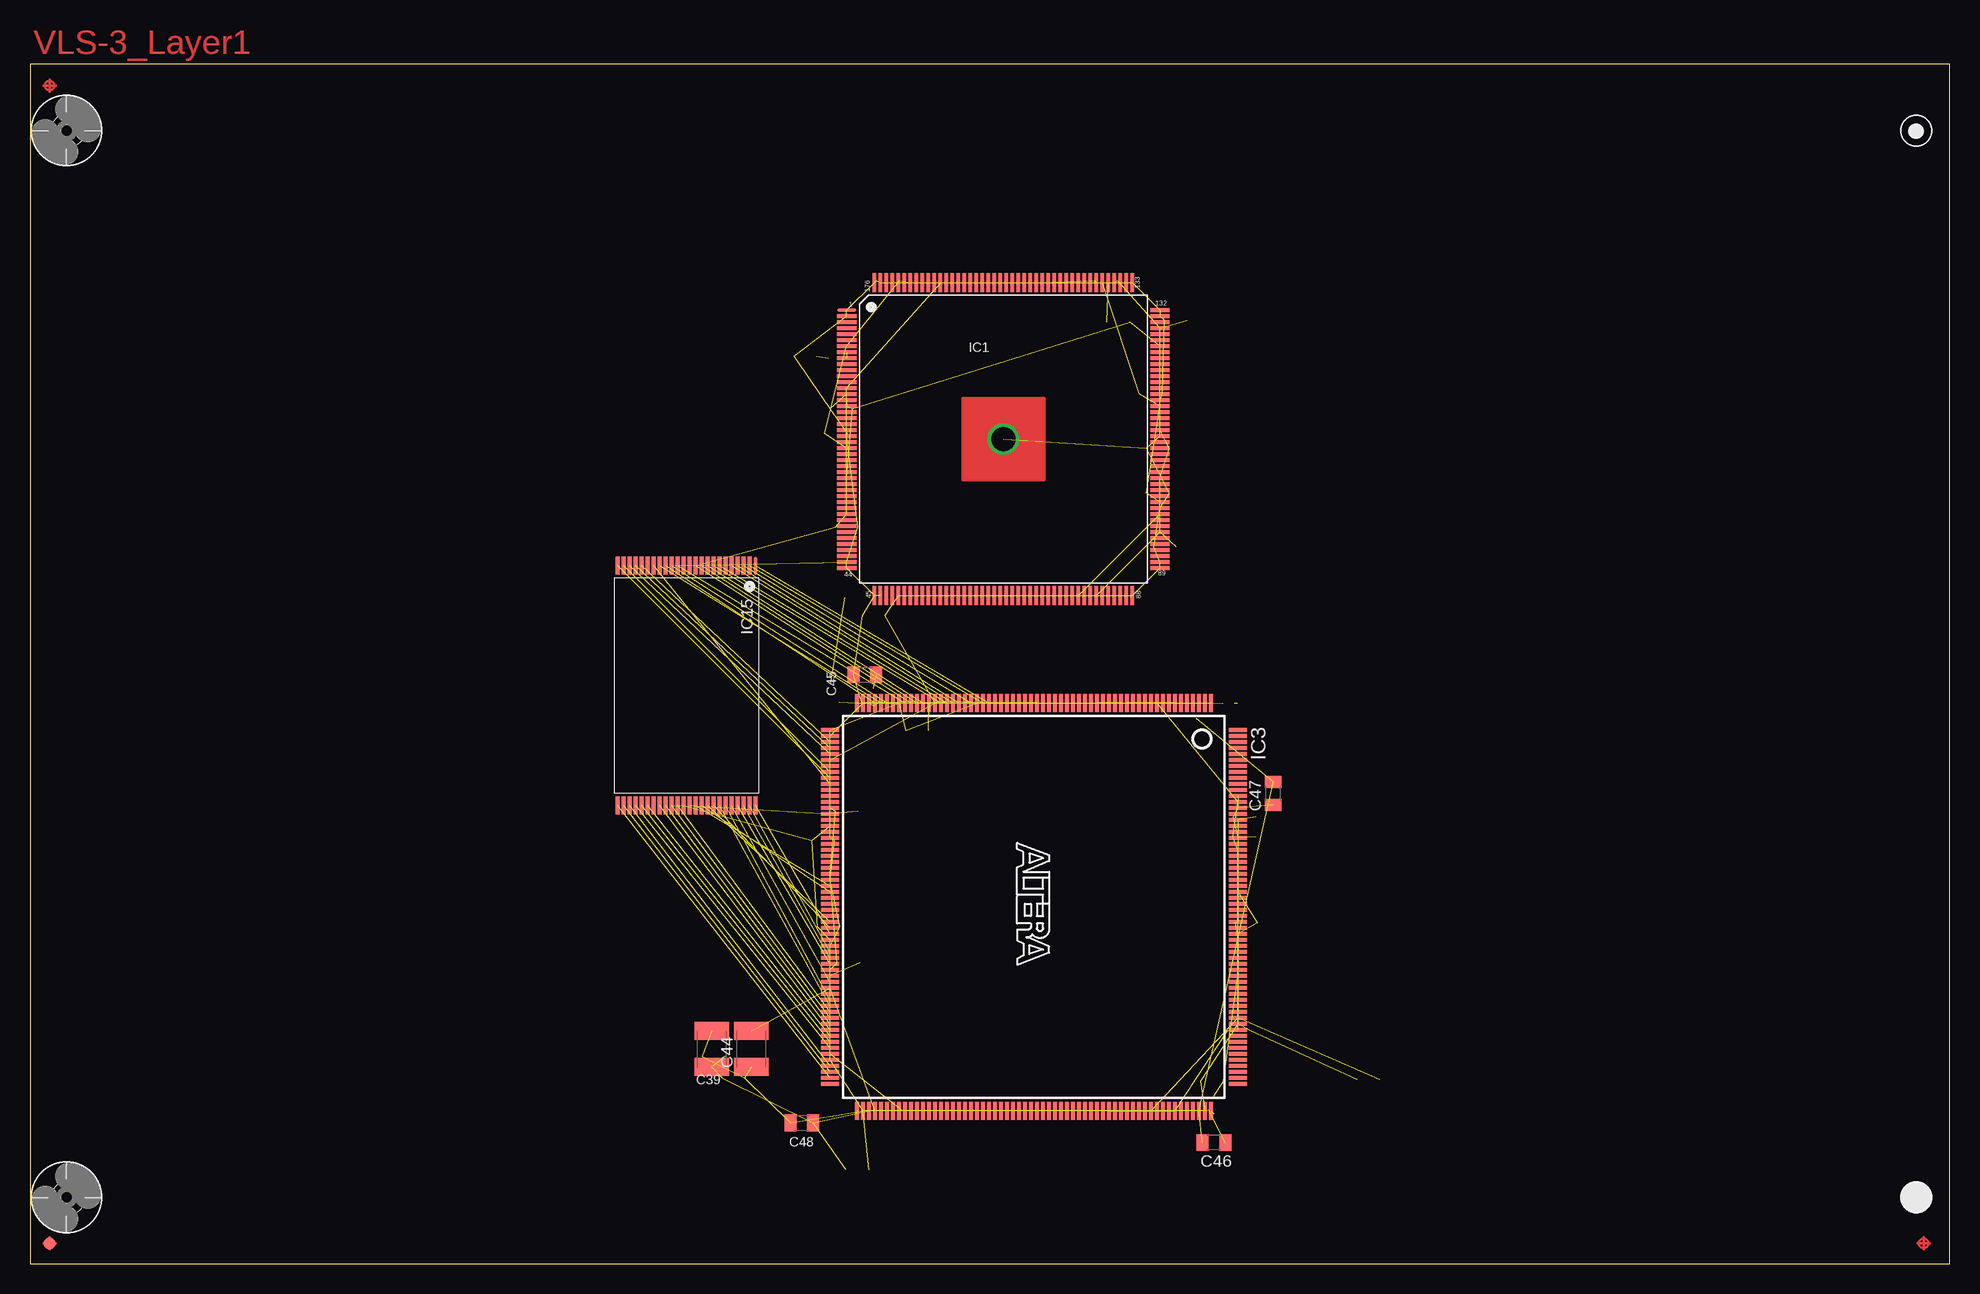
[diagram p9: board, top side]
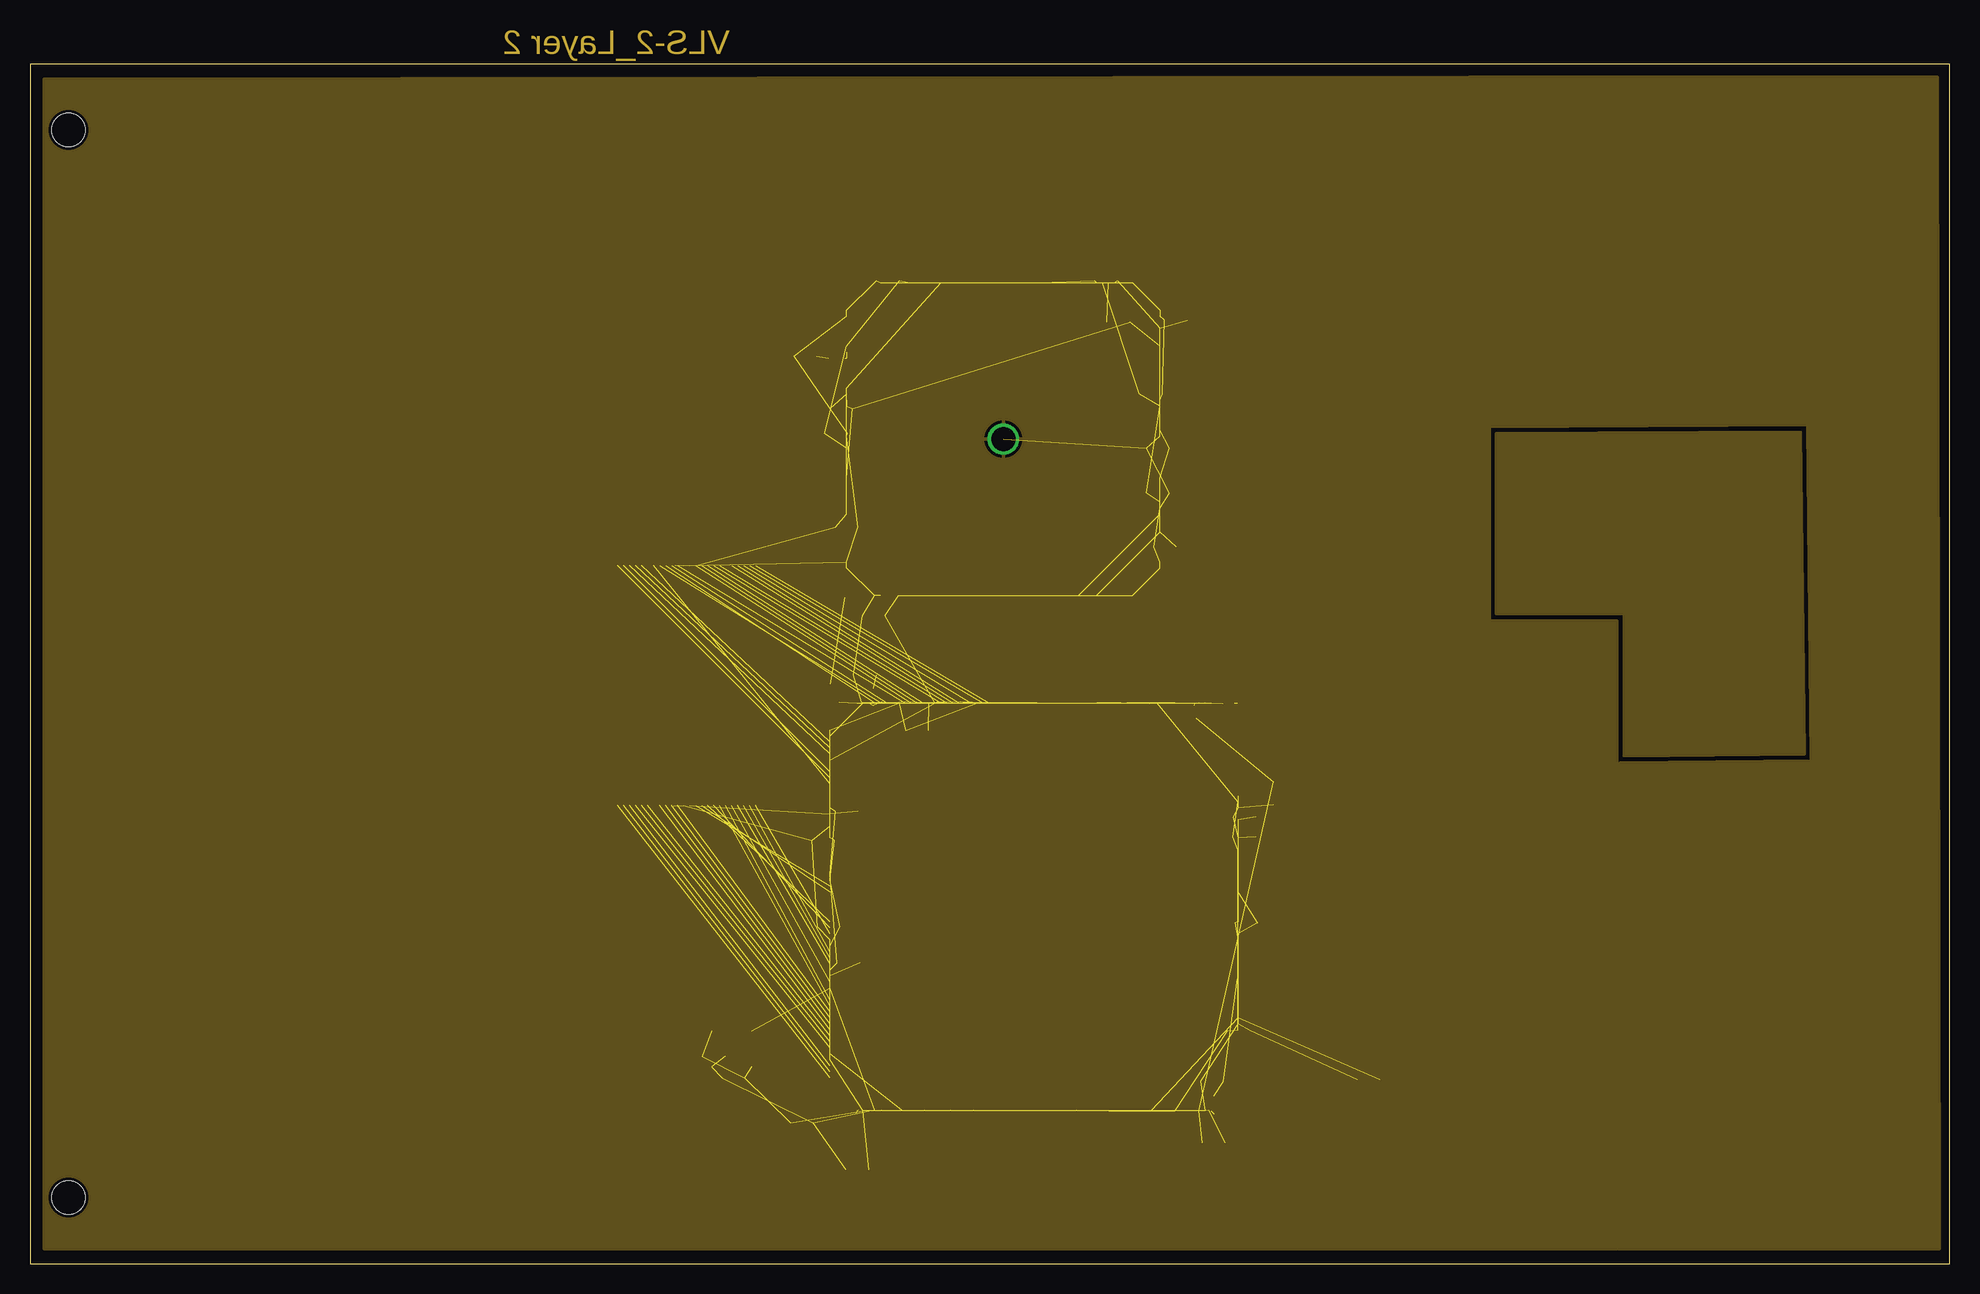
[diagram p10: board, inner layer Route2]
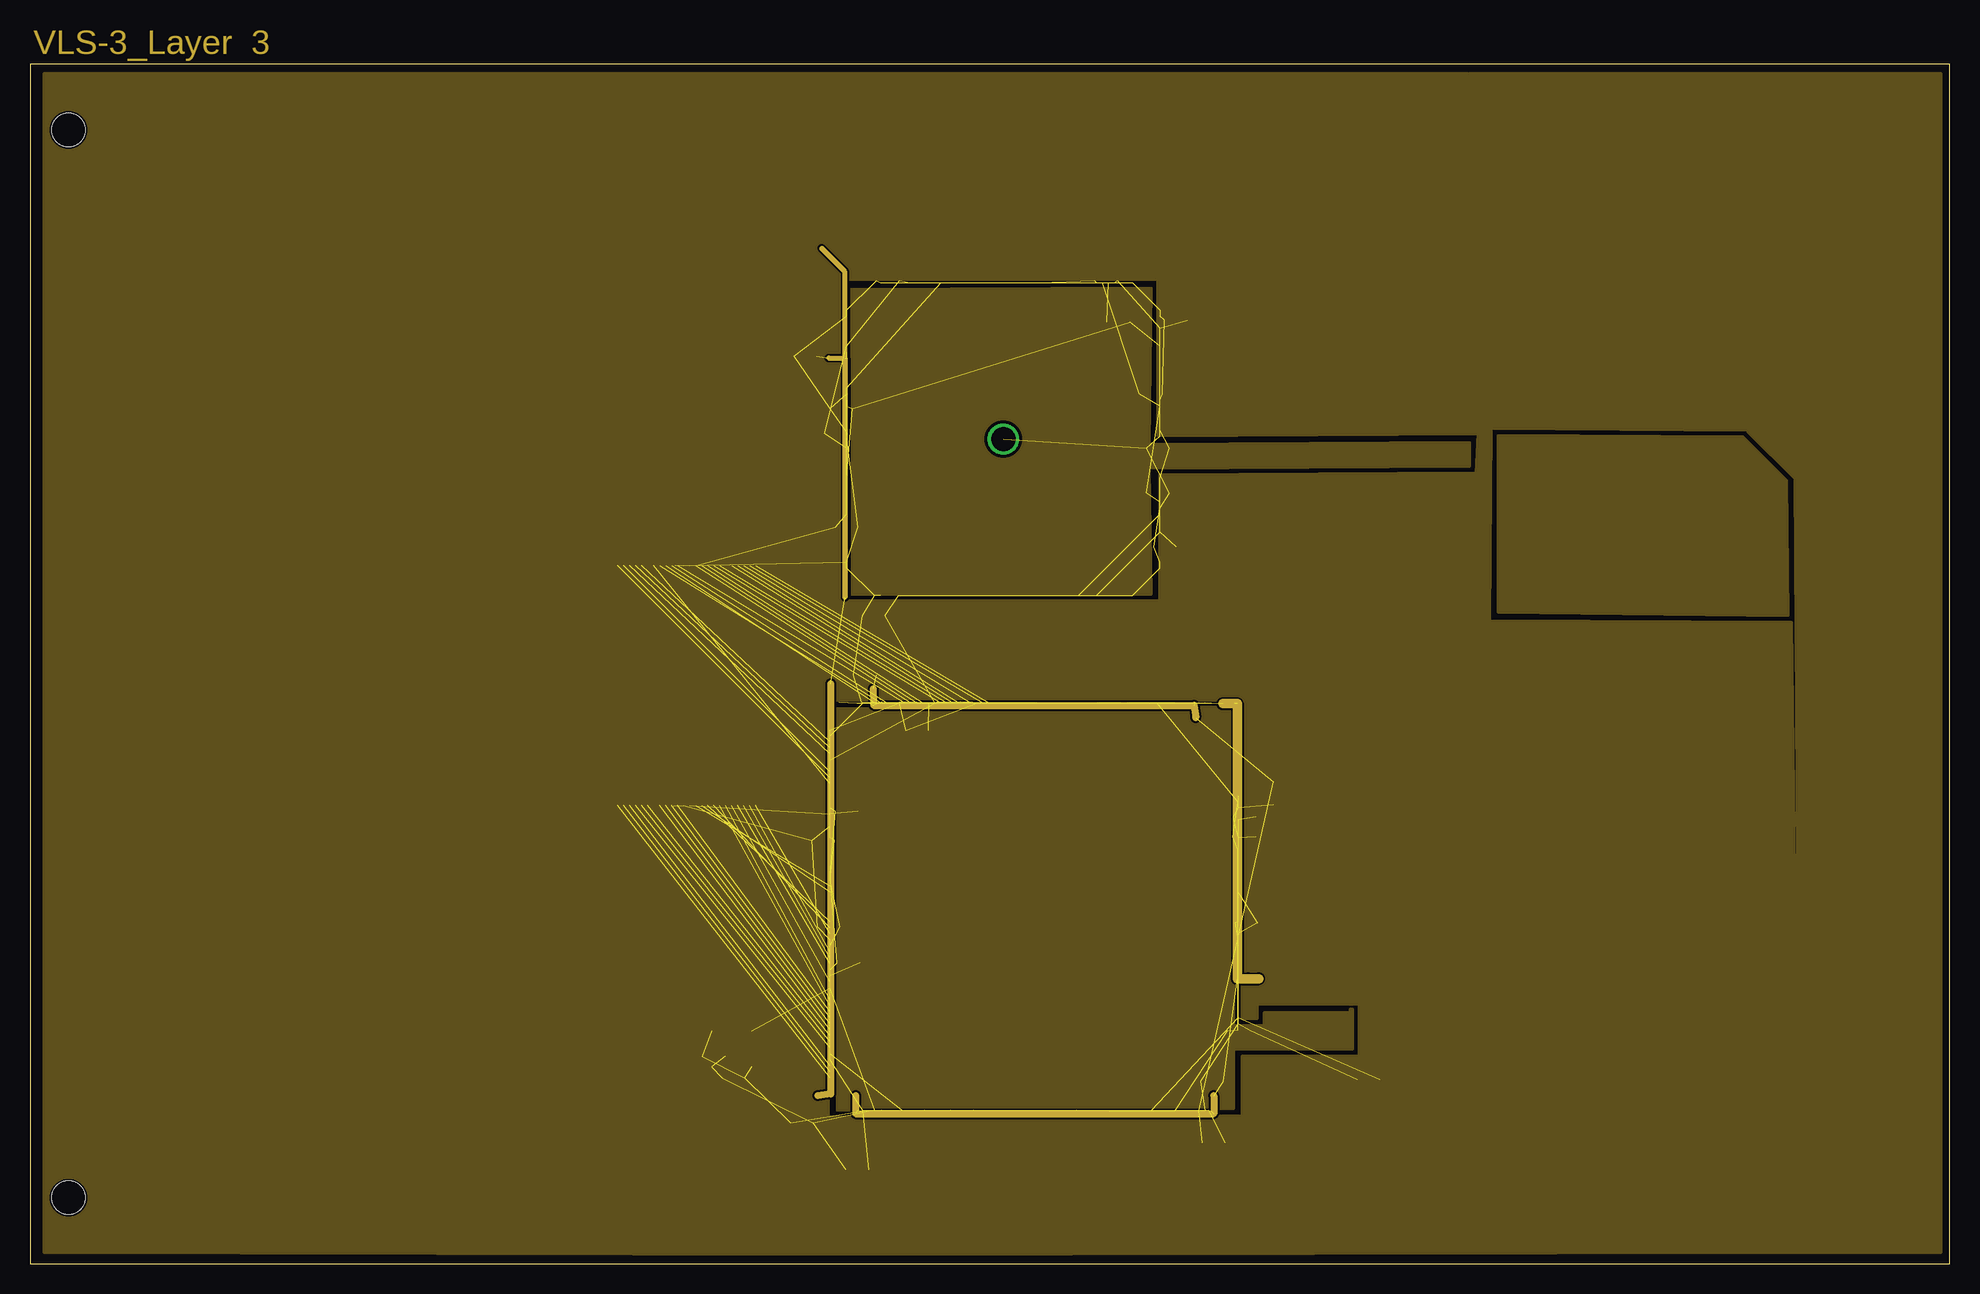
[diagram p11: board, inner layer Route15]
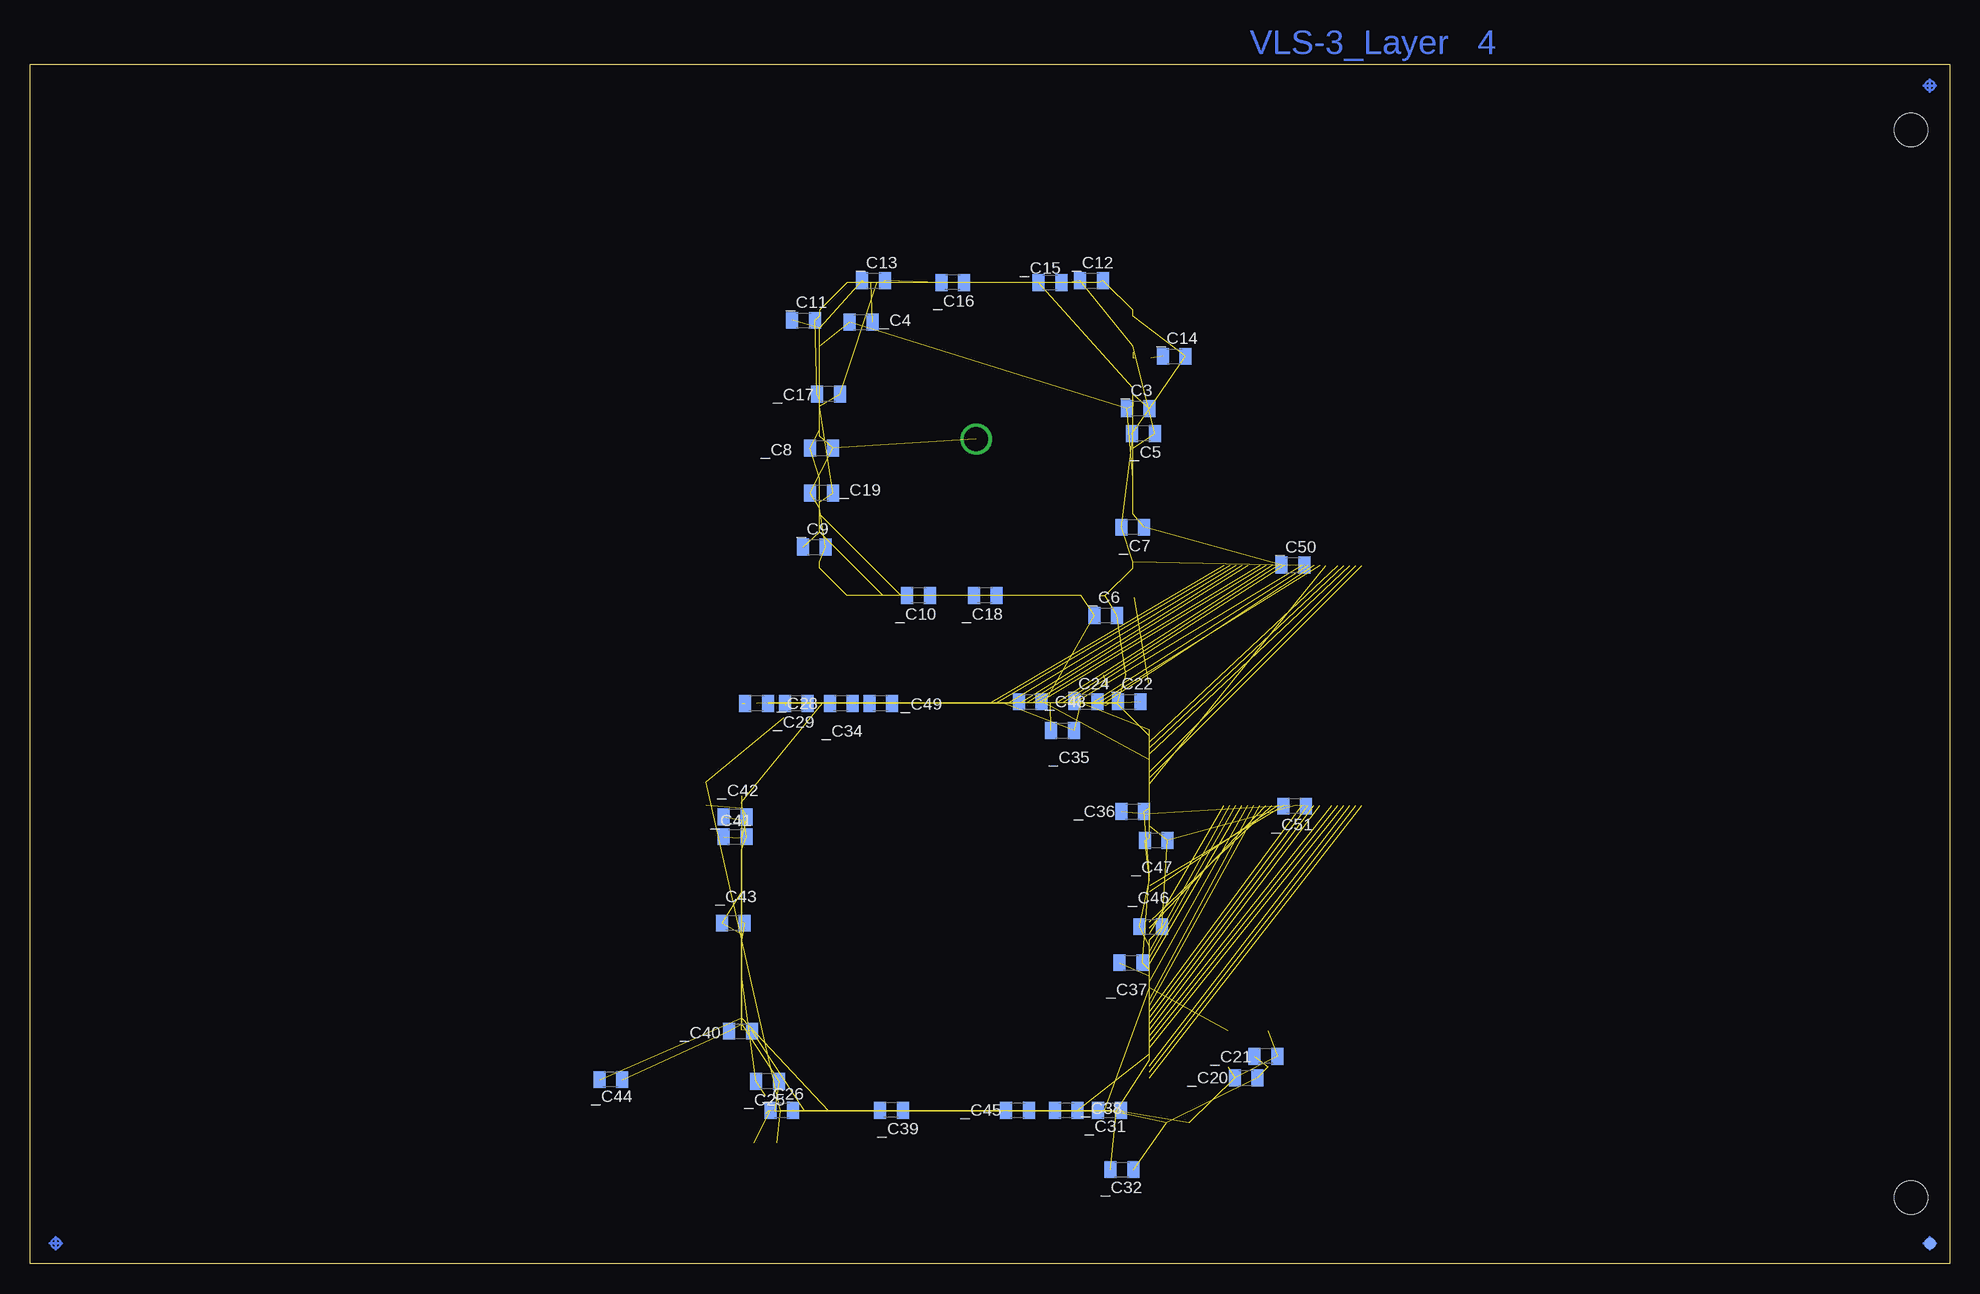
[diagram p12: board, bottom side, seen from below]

Size 160 x 100 mm. Coordinates in mm from the lower left corner, seen from the top.
Copper layers (1*2+15*16): Top 0.035mm / dielectric 1.5mm / Route2 0.035mm / dielectric 0.15mm / Route15 0.035mm / dielectric 0.2mm / Bottom 0.035mm
Design rules "default *": minimum track width 0.15mm, minimum drill 0.3mm, track to track 0.15mm, track to pad 0.15mm, pad to pad 0.15mm, via to via 0.15mm, smd to smd 0.02mm, copper to edge 0.15mm, drill to drill 0.15mm, minimum pad ring 0.25mm, minimum via ring 0.12mm, stop-mask expansion 0.05mm, vias tented up to drill 24mil, thermal gap 10mil

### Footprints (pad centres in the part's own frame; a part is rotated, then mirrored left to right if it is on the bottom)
C0805 = smd 1 x 1.4: 1 -0.95,0; 2 0.95,0
C1210K = smd 1.5 x 2.9: 1 -1.5,0; 2 1.5,0
LQFP-176+GND = smd 1.6 x 0.3: 1 -13.05,10.746; 2 -13.05,10.246; 3 -13.05,9.746; 4 -13.05,9.246; 5 -13.05,8.746; 6 -13.05,8.246; 7 -13.05,7.746; 8 -13.05,7.246; 9 -13.05,6.746; 10 -13.05,6.246; 11 -13.05,5.746; 12 -13.05,5.246; 13 -13.05,4.746; 14 -13.05,4.246; 15 -13.05,3.746; 16 -13.05,3.246; 17 -13.05,2.746; 18 -13.05,2.246; 19 -13.05,1.746; 20 -13.05,1.246; 21 -13.05,0.746; 22 -13.05,0.246; 23 -13.05,-0.254; 24 -13.05,-0.754; 25 -13.05,-1.254; 26 -13.05,-1.754; 27 -13.05,-2.254; 28 -13.05,-2.754; 29 -13.05,-3.254; 30 -13.05,-3.754; 31 -13.05,-4.254; 32 -13.05,-4.754; 33 -13.05,-5.254; 34 -13.05,-5.754; 35 -13.05,-6.254; 36 -13.05,-6.754; 37 -13.05,-7.254; 38 -13.05,-7.754; 39 -13.05,-8.254; 40 -13.05,-8.754; 41 -13.05,-9.254; 42 -13.05,-9.754; 43 -13.05,-10.254; 44 -13.05,-10.754; 89 13.05,-10.75; 90 13.05,-10.25; 91 13.05,-9.75; 92 13.05,-9.25; 93 13.05,-8.75; 94 13.05,-8.25; 95 13.05,-7.75; 96 13.05,-7.25; 97 13.05,-6.75; 98 13.05,-6.25; 99 13.05,-5.75; 100 13.05,-5.25; 101 13.05,-4.75; 102 13.05,-4.25; 103 13.05,-3.75; 104 13.05,-3.25; 105 13.05,-2.75; 106 13.05,-2.25; 107 13.05,-1.75; 108 13.05,-1.25; 109 13.05,-0.75; 110 13.05,-0.25; 111 13.05,0.25; 112 13.05,0.75; 113 13.05,1.25; 114 13.05,1.75; 115 13.05,2.25; 116 13.05,2.75; 117 13.05,3.25; 118 13.05,3.75; 119 13.05,4.25; 120 13.05,4.75; 121 13.05,5.25; 122 13.05,5.75; 123 13.05,6.25; 124 13.05,6.75; 125 13.05,7.25; 126 13.05,7.75; 127 13.05,8.25; 128 13.05,8.75; 129 13.05,9.25; 130 13.05,9.75; 131 13.05,10.25; 132 13.05,10.75 | smd 0.3 x 1.6: 45 -10.75,-13.05; 46 -10.25,-13.05; 47 -9.75,-13.05; 48 -9.25,-13.05; 49 -8.75,-13.05; 50 -8.25,-13.05; 51 -7.75,-13.05; 52 -7.25,-13.05; 53 -6.75,-13.05; 54 -6.25,-13.05; 55 -5.75,-13.05; 56 -5.25,-13.05; 57 -4.75,-13.05; 58 -4.25,-13.05; 59 -3.75,-13.05; 60 -3.25,-13.05; 61 -2.75,-13.05; 62 -2.25,-13.05; 63 -1.75,-13.05; 64 -1.25,-13.05; 65 -0.75,-13.05; 66 -0.25,-13.05; 67 0.25,-13.05; 68 0.75,-13.05; 69 1.25,-13.05; 70 1.75,-13.05; 71 2.25,-13.05; 72 2.75,-13.05; 73 3.25,-13.05; 74 3.75,-13.05; 75 4.25,-13.05; 76 4.75,-13.05; 77 5.25,-13.05; 78 5.75,-13.05; 79 6.25,-13.05; 80 6.75,-13.05; 81 7.25,-13.05; 82 7.75,-13.05; 83 8.25,-13.05; 84 8.75,-13.05; 85 9.25,-13.05; 86 9.75,-13.05; 87 10.25,-13.05; 88 10.75,-13.05; 133 10.75,13.05; 134 10.25,13.05; 135 9.75,13.05; 136 9.25,13.05; 137 8.75,13.05; 138 8.25,13.05; 139 7.75,13.05; 140 7.25,13.05; 141 6.75,13.05; 142 6.25,13.05; 143 5.75,13.05; 144 5.25,13.05; 145 4.75,13.05; 146 4.25,13.05; 147 3.75,13.05; 148 3.25,13.05; 149 2.75,13.05; 150 2.25,13.05; 151 1.75,13.05; 152 1.25,13.05; 153 0.75,13.05; 154 0.25,13.05; 155 -0.25,13.05; 156 -0.75,13.05; 157 -1.25,13.05; 158 -1.75,13.05; 159 -2.25,13.05; 160 -2.75,13.05; 161 -3.25,13.05; 162 -3.75,13.05; 163 -4.25,13.05; 164 -4.75,13.05; 165 -5.25,13.05; 166 -5.75,13.05; 167 -6.25,13.05; 168 -6.75,13.05; 169 -7.25,13.05; 170 -7.75,13.05; 171 -8.25,13.05; 172 -8.75,13.05; 173 -9.25,13.05; 174 -9.75,13.05; 175 -10.25,13.05; 176 -10.75,13.05 | drill 2: CENTER 0,0
PQFP240 = smd 1.5 x 0.32: 1 -17,14.75; 2 -17,14.25; 3 -17,13.75; 4 -17,13.25; 5 -17,12.75; 6 -17,12.25; 7 -17,11.75; 8 -17,11.25; 9 -17,10.75; 10 -17,10.25; 11 -17,9.75; 12 -17,9.25; 13 -17,8.75; 14 -17,8.25; 15 -17,7.75; 16 -17,7.25; 17 -17,6.75; 18 -17,6.25; 19 -17,5.75; 20 -17,5.25; 21 -17,4.75; 22 -17,4.25; 23 -17,3.75; 24 -17,3.25; 25 -17,2.75; 26 -17,2.25; 27 -17,1.75; 28 -17,1.25; 29 -17,0.75; 30 -17,0.25; 31 -17,-0.25; 32 -17,-0.75; 33 -17,-1.25; 34 -17,-1.75; 35 -17,-2.25; 36 -17,-2.75; 37 -17,-3.25; 38 -17,-3.75; 39 -17,-4.25; 40 -17,-4.75; 41 -17,-5.25; 42 -17,-5.75; 43 -17,-6.25; 44 -17,-6.75; 45 -17,-7.25; 46 -17,-7.75; 47 -17,-8.25; 48 -17,-8.75; 49 -17,-9.25; 50 -17,-9.75; 51 -17,-10.25; 52 -17,-10.75; 53 -17,-11.25; 54 -17,-11.75; 55 -17,-12.25; 56 -17,-12.75; 57 -17,-13.25; 58 -17,-13.75; 59 -17,-14.25; 60 -17,-14.75; 121 17,-14.75; 122 17,-14.25; 123 17,-13.75; 124 17,-13.25; 125 17,-12.75; 126 17,-12.25; 127 17,-11.75; 128 17,-11.25; 129 17,-10.75; 130 17,-10.25; 131 17,-9.75; 132 17,-9.25; 133 17,-8.75; 134 17,-8.25; 135 17,-7.75; 136 17,-7.25; 137 17,-6.75; 138 17,-6.25; 139 17,-5.75; 140 17,-5.25; 141 17,-4.75; 142 17,-4.25; 143 17,-3.75; 144 17,-3.25; 145 17,-2.75; 146 17,-2.25; 147 17,-1.75; 148 17,-1.25; 149 17,-0.75; 150 17,-0.25; 151 17,0.25; 152 17,0.75; 153 17,1.25; 154 17,1.75; 155 17,2.25; 156 17,2.75; 157 17,3.25; 158 17,3.75; 159 17,4.25; 160 17,4.75; 161 17,5.25; 162 17,5.75; 163 17,6.25; 164 17,6.75; 165 17,7.25; 166 17,7.75; 167 17,8.25; 168 17,8.75; 169 17,9.25; 170 17,9.75; 171 17,10.25; 172 17,10.75; 173 17,11.25; 174 17,11.75; 175 17,12.25; 176 17,12.75; 177 17,13.25; 178 17,13.75; 179 17,14.25; 180 17,14.75 | smd 0.32 x 1.5: 61 -14.75,-17; 62 -14.25,-17; 63 -13.75,-17; 64 -13.25,-17; 65 -12.75,-17; 66 -12.25,-17; 67 -11.75,-17; 68 -11.25,-17; 69 -10.75,-17; 70 -10.25,-17; 71 -9.75,-17; 72 -9.25,-17; 73 -8.75,-17; 74 -8.25,-17; 75 -7.75,-17; 76 -7.25,-17; 77 -6.75,-17; 78 -6.25,-17; 79 -5.75,-17; 80 -5.25,-17; 81 -4.75,-17; 82 -4.25,-17; 83 -3.75,-17; 84 -3.25,-17; 85 -2.75,-17; 86 -2.25,-17; 87 -1.75,-17; 88 -1.25,-17; 89 -0.75,-17; 90 -0.25,-17; 91 0.25,-17; 92 0.75,-17; 93 1.25,-17; 94 1.75,-17; 95 2.25,-17; 96 2.75,-17; 97 3.25,-17; 98 3.75,-17; 99 4.25,-17; 100 4.75,-17; 101 5.25,-17; 102 5.75,-17; 103 6.25,-17; 104 6.75,-17; 105 7.25,-17; 106 7.75,-17; 107 8.25,-17; 108 8.75,-17; 109 9.25,-17; 110 9.75,-17; 111 10.25,-17; 112 10.75,-17; 113 11.25,-17; 114 11.75,-17; 115 12.25,-17; 116 12.75,-17; 117 13.25,-17; 118 13.75,-17; 119 14.25,-17; 120 14.75,-17; 181 14.75,17; 182 14.25,17; 183 13.75,17; 184 13.25,17; 185 12.75,17; 186 12.25,17; 187 11.75,17; 188 11.25,17; 189 10.75,17; 190 10.25,17; 191 9.75,17; 192 9.25,17; 193 8.75,17; 194 8.25,17; 195 7.75,17; 196 7.25,17; 197 6.75,17; 198 6.25,17; 199 5.75,17; 200 5.25,17; 201 4.75,17; 202 4.25,17; 203 3.75,17; 204 3.25,17; 205 2.75,17; 206 2.25,17; 207 1.75,17; 208 1.25,17; 209 0.75,17; 210 0.25,17; 211 -0.25,17; 212 -0.75,17; 213 -1.25,17; 214 -1.75,17; 215 -2.25,17; 216 -2.75,17; 217 -3.25,17; 218 -3.75,17; 219 -4.25,17; 220 -4.75,17; 221 -5.25,17; 222 -5.75,17; 223 -6.25,17; 224 -6.75,17; 225 -7.25,17; 226 -7.75,17; 227 -8.25,17; 228 -8.75,17; 229 -9.25,17; 230 -9.75,17; 231 -10.25,17; 232 -10.75,17; 233 -11.25,17; 234 -11.75,17; 235 -12.25,17; 236 -12.75,17; 237 -13.25,17; 238 -13.75,17; 239 -14.25,17; 240 -14.75,17
TSOP1-12X20 = smd 1.5 x 0.3: 1 -10,5.75; 2 -10,5.25; 3 -10,4.75; 4 -10,4.25; 5 -10,3.75; 6 -10,3.25; 7 -10,2.75; 8 -10,2.25; 9 -10,1.75; 10 -10,1.25; 11 -10,0.75; 12 -10,0.25; 13 -10,-0.25; 14 -10,-0.75; 15 -10,-1.25; 16 -10,-1.75; 17 -10,-2.25; 18 -10,-2.75; 19 -10,-3.25; 20 -10,-3.75; 21 -10,-4.25; 22 -10,-4.75; 23 -10,-5.25; 24 -10,-5.75; 25 10,-5.75; 26 10,-5.25; 27 10,-4.75; 28 10,-4.25; 29 10,-3.75; 30 10,-3.25; 31 10,-2.75; 32 10,-2.25; 33 10,-1.75; 34 10,-1.25; 35 10,-0.75; 36 10,-0.25; 37 10,0.25; 38 10,0.75; 39 10,1.25; 40 10,1.75; 41 10,2.25; 42 10,2.75; 43 10,3.25; 44 10,3.75; 45 10,4.25; 46 10,4.75; 47 10,5.25; 48 10,5.75
PCB = smd 1 x 1 bottom: S-0.0 0,0 | smd 1 x 1: T-0.0 0,0
EURO = hole 2.794: 1.575,3.81; 1.575,92.812

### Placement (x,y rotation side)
_C3  67.63,71.3 0 bottom
_C4  90.73,78.5 0 bottom
_C5  67.18,69.2 180 bottom
_C6  70.33,54.05 0 bottom
_C7  68.08,61.4 180 bottom
_C8  94.03,68 0 bottom
_C9  94.63,59.75 0 bottom
_C10  85.93,55.7 180 bottom
_C11  95.53,78.65 0 bottom
_C12  71.53,81.95 0 bottom
_C13  89.68,81.95 0 bottom
_C14  64.63,75.65 0 bottom
_C15  74.98,81.8 0 bottom
_C16  83.08,81.8 180 bottom
_C17  93.43,72.5 180 bottom
_C18  80.38,55.7 180 bottom
_C19  94.03,64.25 180 bottom
_C20  58.63,15.5 0 bottom
_C21  56.98,17.3 180 bottom
_C22  68.38,46.85 0 bottom
_C24  71.98,46.85 0 bottom
_C25  98.53,15.2 180 bottom
_C26  97.33,12.8 0 bottom
_C28  99.43,46.7 180 bottom
_C29  96.13,46.7 180 bottom
_C31  70.03,12.8 0 bottom
_C32  68.98,7.85 0 bottom
_C34  92.38,46.7 180 bottom
_C35  73.93,44.45 0 bottom
_C36  68.08,37.7 0 bottom
_C37  68.23,25.1 0 bottom
_C38  73.63,12.8 0 bottom
_C39  88.18,12.8 180 bottom
_C40  100.78,19.4 0 bottom
_C41  101.23,35.6 0 bottom
_C42  101.23,37.25 180 bottom
_C43  101.38,28.4 180 bottom
_C44  111.58,15.35 180 bottom
_C45  77.68,12.8 0 bottom
_C46  66.58,28.1 0 bottom
_C47  66.13,35.3 0 bottom
_C48  76.63,46.85 0 bottom
_C49  89.08,46.7 180 bottom
_C50  54.73,58.25 0 bottom
_C51  54.58,38.15 180 bottom
C39  56.83,17.9 270 top
C44  60.13,17.9 90 top
C45  69.58,49.1 0 top
C46  98.68,10.1 180 top
C47  103.63,39.2 90 top
C48  64.33,11.75 0 top
IC1  81.13,68.75 0 top
IC3  83.68,29.75 270 top
IC15  54.73,48.2 270 top
PCB  1.63,1.7 0 top
U$1  [EURO]  1.63,1.7 0 top

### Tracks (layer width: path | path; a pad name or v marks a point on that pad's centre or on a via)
1V2  (25 unrouted)
  pour Route15 (isolate 0.15): 67.18,46.25 100.33,46.4 100.33,19.85 102.88,19.85 102.88,20.9 110.08,20.9 110.08,21.2 110.23,21.2 110.23,17.9 100.33,17.9 100.33,12.95 67.33,12.8
1V2_PLL  (9 unrouted)
  Route15 0.6: 98.68,14 98.68,12.5 68.83,12.5 68.83,14
  Route15 0.8: 99.43,46.7 100.63,46.7 100.63,24.2 100.63,23.75 101.53,23.75 102.43,23.75
1V4  (15 unrouted)
  pour Route15 (isolate 0.254): 68.38,81.2 93.43,81.35 93.28,68.3 119.98,68.45 119.98,66.5 93.28,66.35 93.43,55.85 68.38,55.85
1V8  (5 unrouted)
2V5  (4 unrouted)
  Route15 0.4: 66.58,75.5 67.93,75.5 67.93,55.55 67.93,82.7 65.98,84.65
  Route15 0.6: 66.73,48.35 66.73,14.15 65.68,14
2V5_VCCA  (15 unrouted)
  Route15 0.6: 70.28,47.95 70.33,46.55 97.03,46.55 97.18,45.5
3V3  (57 unrouted)
  pour Route15 (isolate 0.15): 1.18,99.2 119.83,99.2 119.83,95.45 93.88,95.45 93.88,82.1 67.48,82.1 67.48,55.25 94.18,55.25 94.18,65.75 120.58,65.9 120.73,69.2 94.03,69.05 94.03,95.3 119.98,95.3 119.98,99.2 159.28,99.2 159.28,0.95 147.58,0.95 147.13,65.45 143.23,69.35 143.23,69.5 121.78,69.65 121.63,53.6 146.83,53.45 147.43,0.95 66.73,0.8 66.73,12.2 101.08,12.35 101.08,17.3 110.83,17.3 110.83,21.65 102.28,21.65 102.28,20.45 101.08,20.45 101.08,47 66.43,47 66.58,0.8 1.18,0.95
3V3A
  pour Route15 (isolate 0.254): 122.38,69.05 142.63,68.9 142.78,68.9 146.38,65.3 146.53,54.05 122.38,54.35
GND  (125 unrouted)
  pour Route2 (isolate 0.254): 1.18,98.75 119.98,98.9 158.98,98.9 159.13,1.25 132.43,1.25 132.58,41.75 148.48,41.9 148.18,69.95 121.63,69.8 121.63,53.6 132.28,53.6 132.28,1.25 1.18,1.25
GNDA
  pour Route2 (isolate 0.15): 122.23,69.2 147.58,69.35 147.88,42.5 132.88,42.35 132.88,54.2 122.23,54.2
RA0  (1 unrouted)
RA1  (1 unrouted)
RA2  (1 unrouted)
RA3  (1 unrouted)
RA4  (1 unrouted)
RA5  (1 unrouted)
RA6  (1 unrouted)
RA7  (1 unrouted)
RA8  (1 unrouted)
RA9  (1 unrouted)
RA10  (1 unrouted)
RA11  (1 unrouted)
RA12  (1 unrouted)
RA13  (1 unrouted)
RA14  (1 unrouted)
RA15  (1 unrouted)
RA16  (1 unrouted)
RA17  (1 unrouted)
RA18  (1 unrouted)
RA19  (1 unrouted)
RCS  (1 unrouted)
RD0  (1 unrouted)
RD1  (1 unrouted)
RD2  (1 unrouted)
RD3  (1 unrouted)
RD4  (1 unrouted)
RD5  (1 unrouted)
RD6  (1 unrouted)
RD7  (1 unrouted)
RD8  (1 unrouted)
RD9  (1 unrouted)
RD10  (1 unrouted)
RD11  (1 unrouted)
RD12  (1 unrouted)
RD13  (1 unrouted)
RD14  (1 unrouted)
RD15  (1 unrouted)
RLB  (1 unrouted)
ROE  (1 unrouted)
RUB  (1 unrouted)
RWE  (1 unrouted)

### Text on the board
Top: VLS-3_Layer1
Route2: VLS-2_Layer 2
Route15: VLS-3_Layer 3
Bottom: VLS-3_Layer 4
tStop: VLS-2_Stop S1
bStop: VLS-2_Stop S 2
tCream: VLS-2_Cream CR1
bCream: VLS-2_Cream CR 2
Document: rot gelb | grün gelb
